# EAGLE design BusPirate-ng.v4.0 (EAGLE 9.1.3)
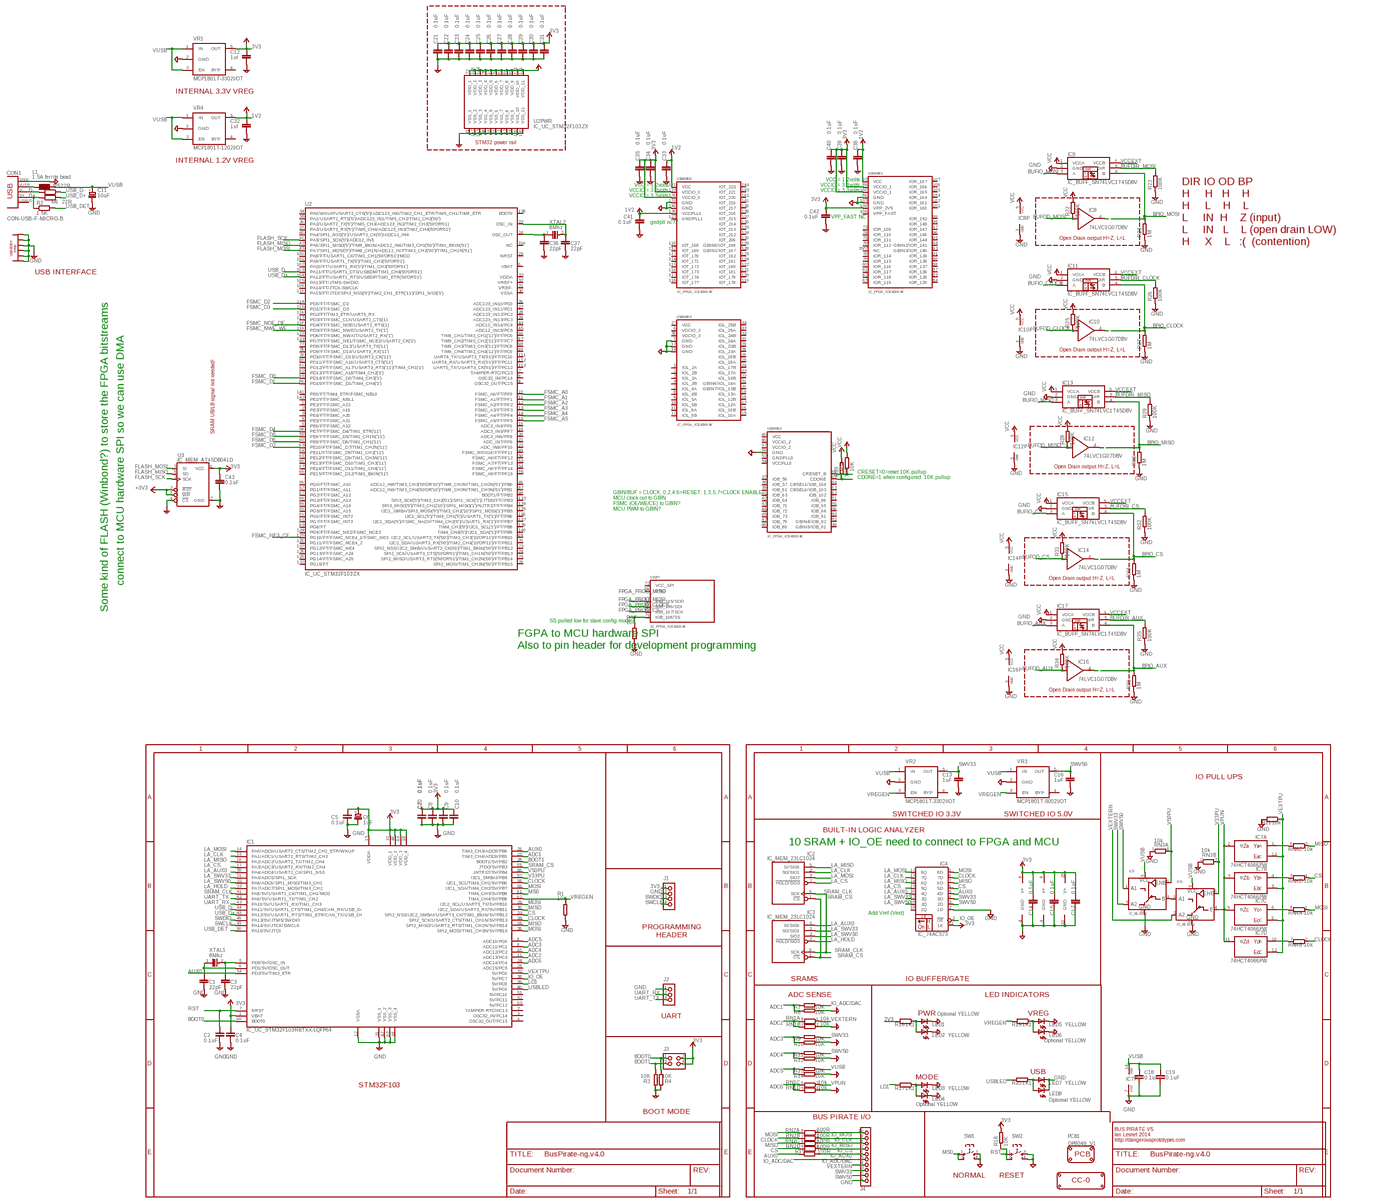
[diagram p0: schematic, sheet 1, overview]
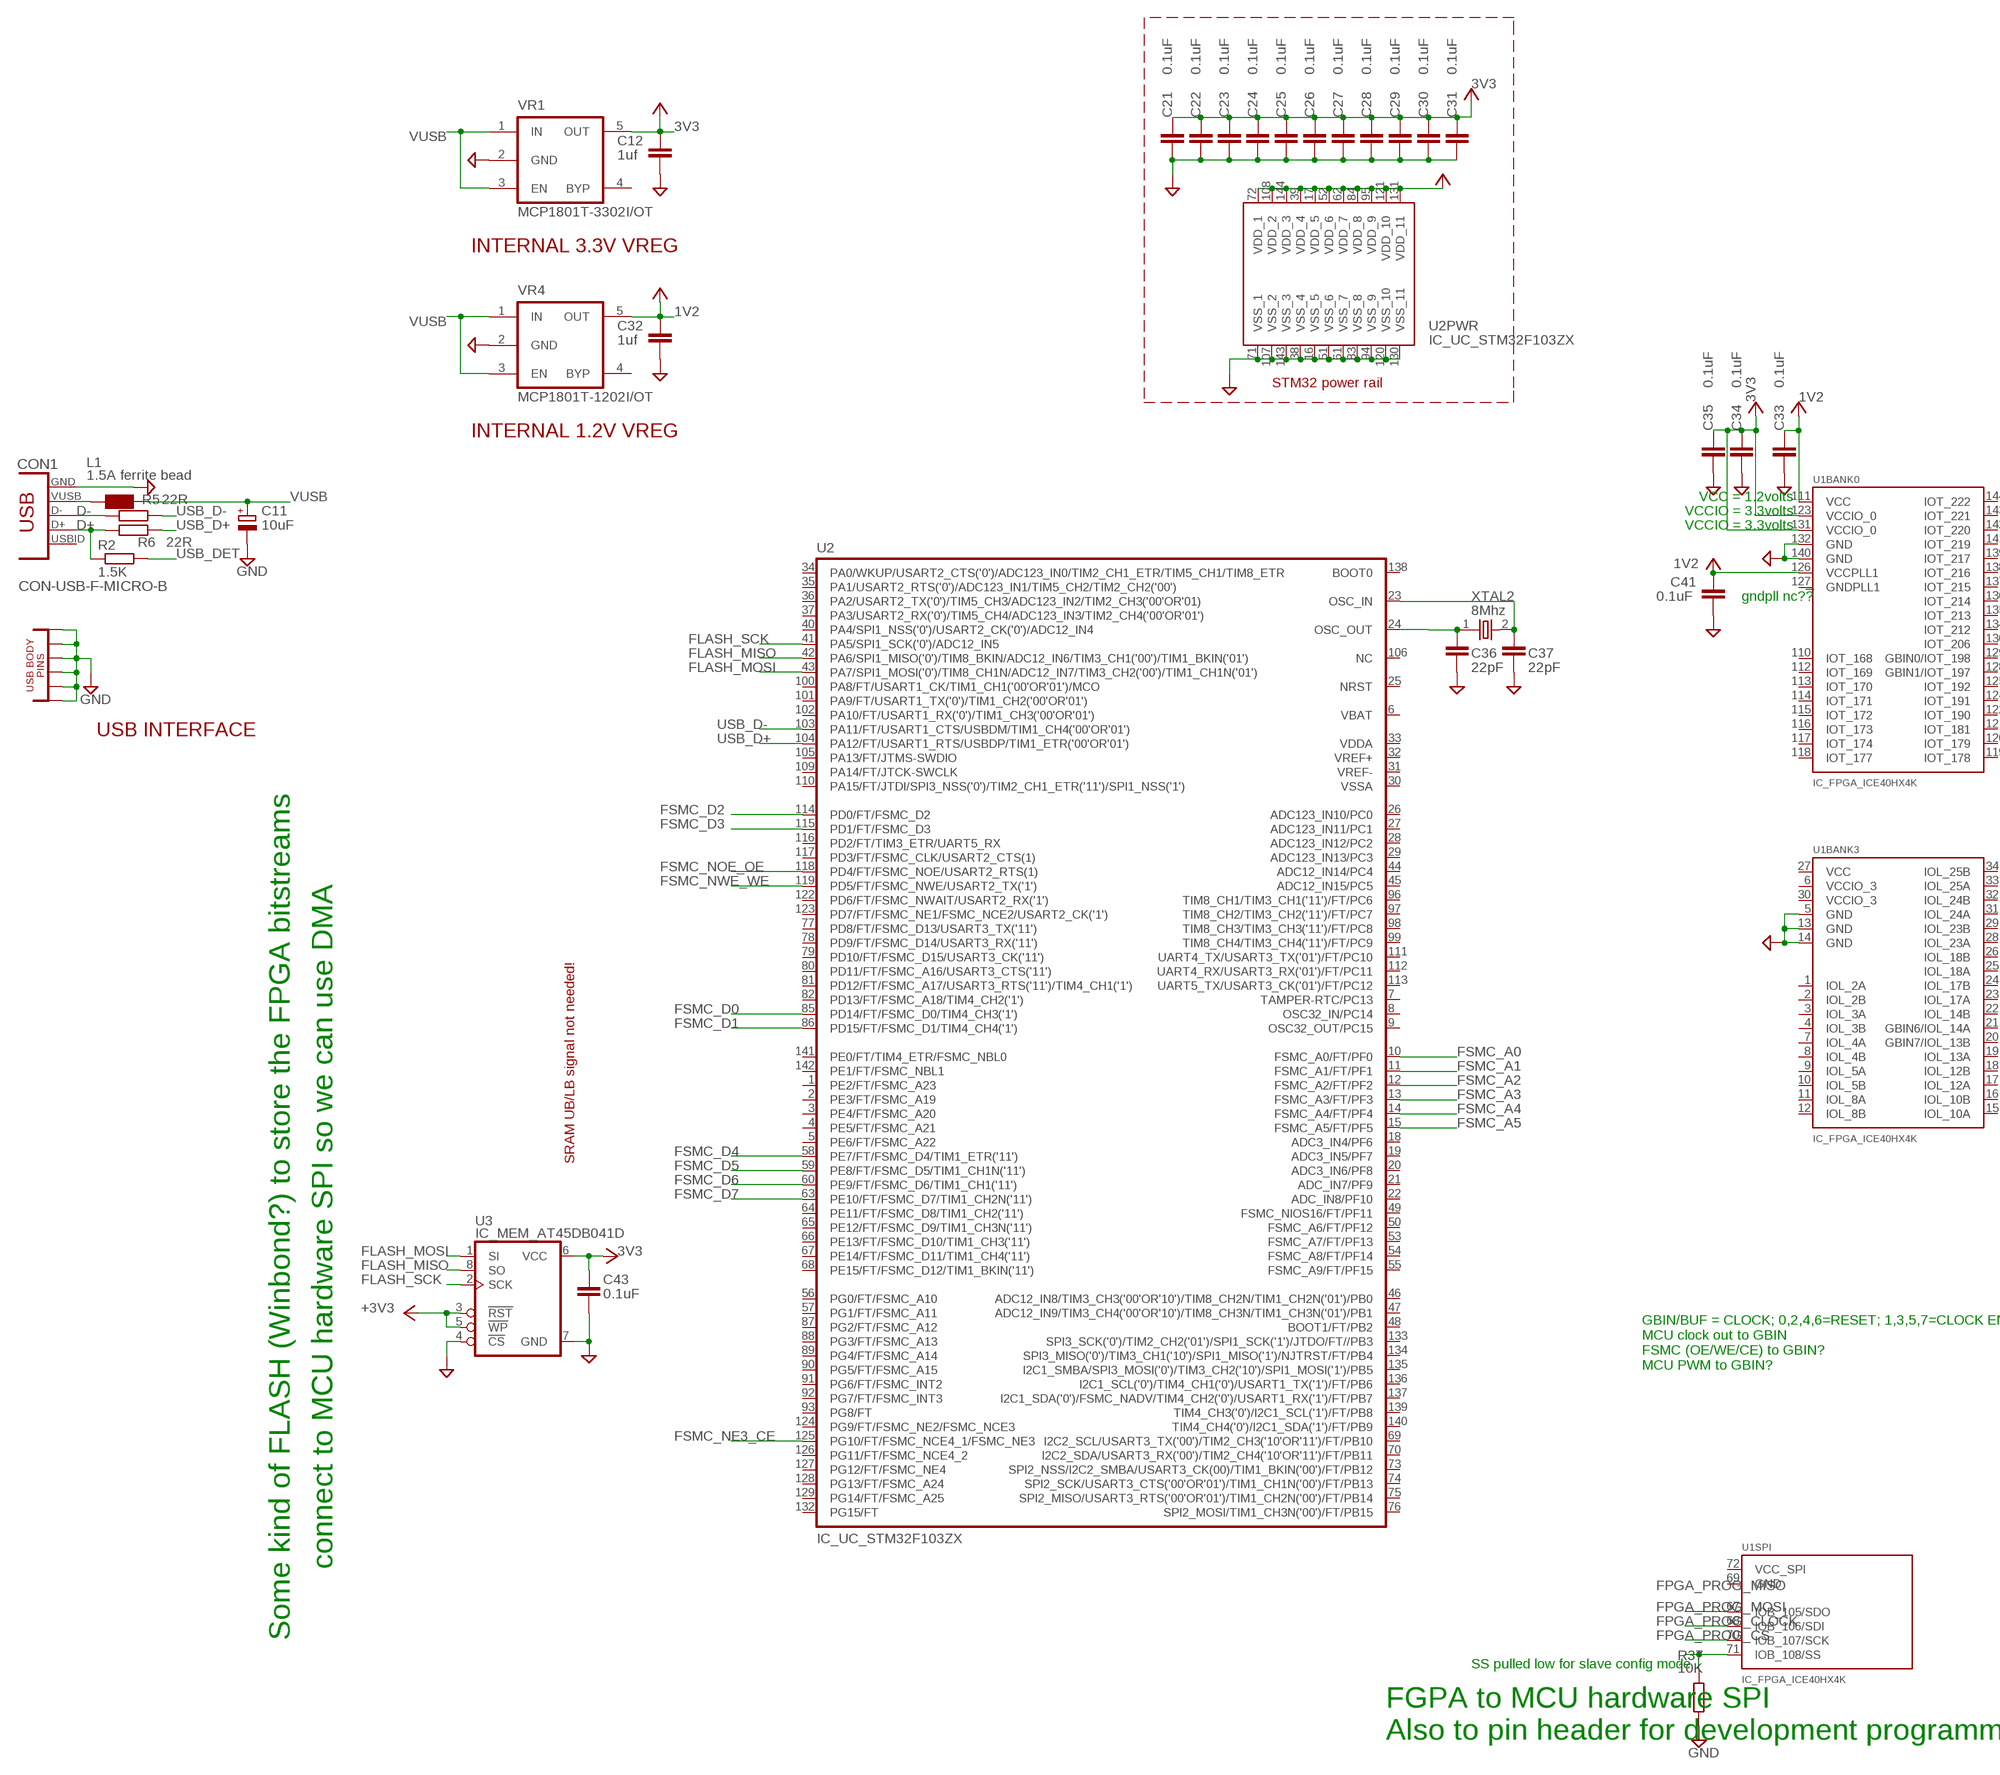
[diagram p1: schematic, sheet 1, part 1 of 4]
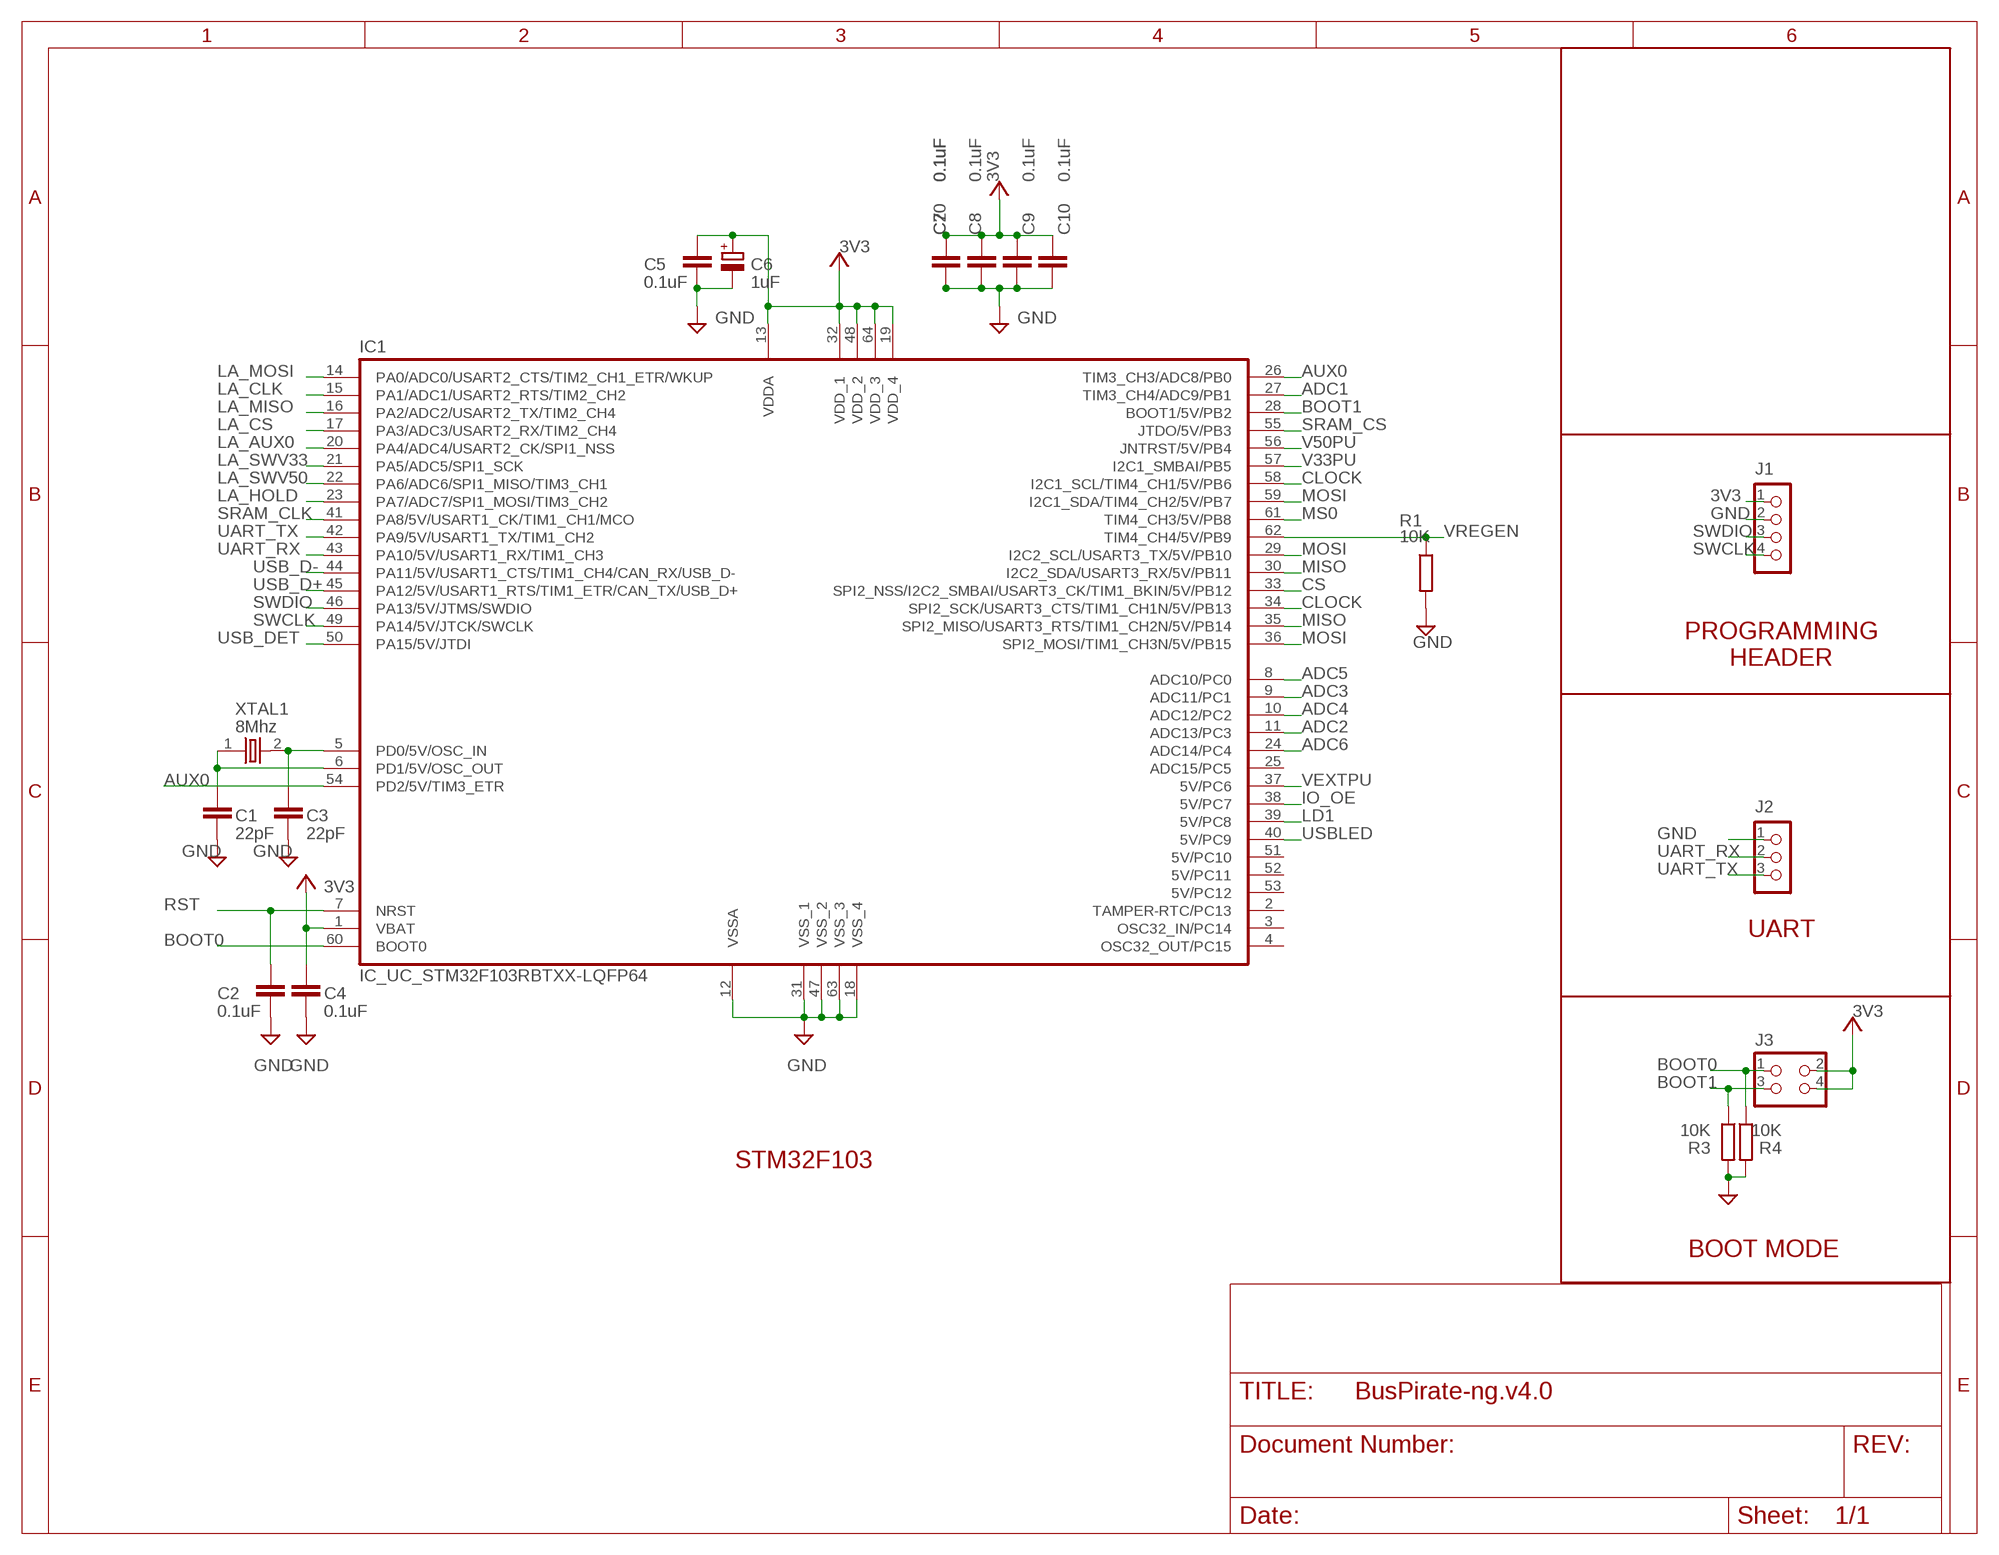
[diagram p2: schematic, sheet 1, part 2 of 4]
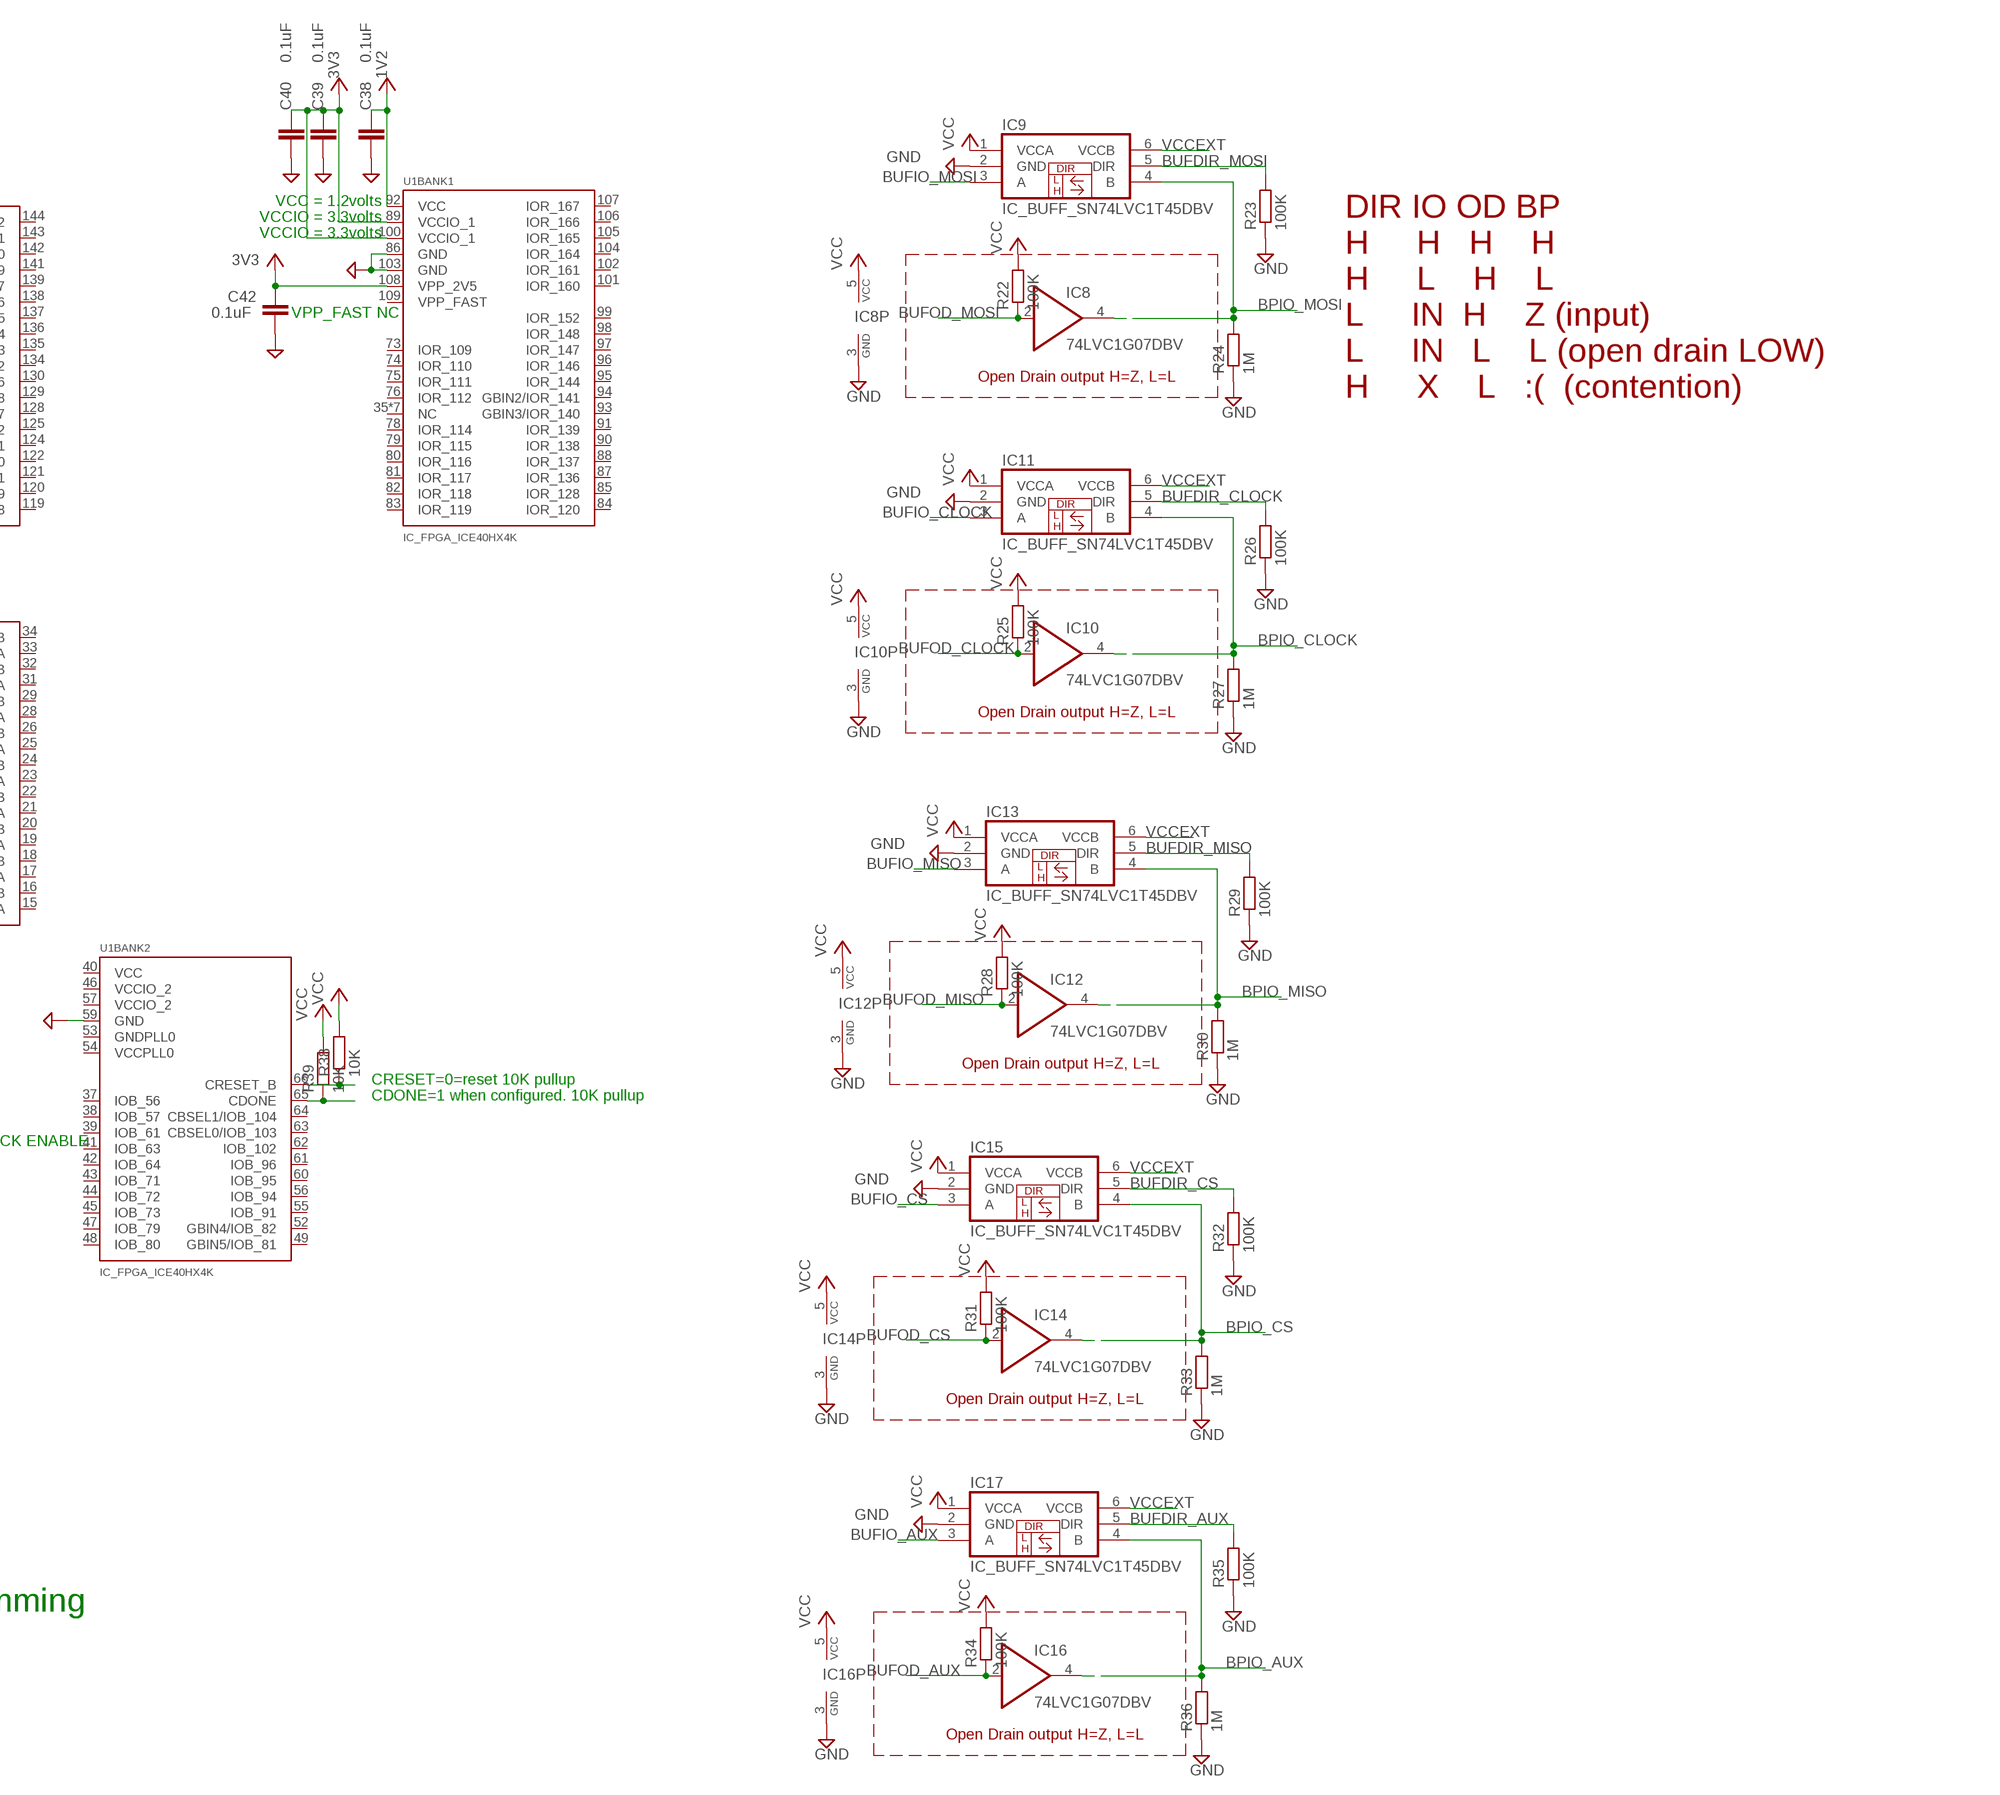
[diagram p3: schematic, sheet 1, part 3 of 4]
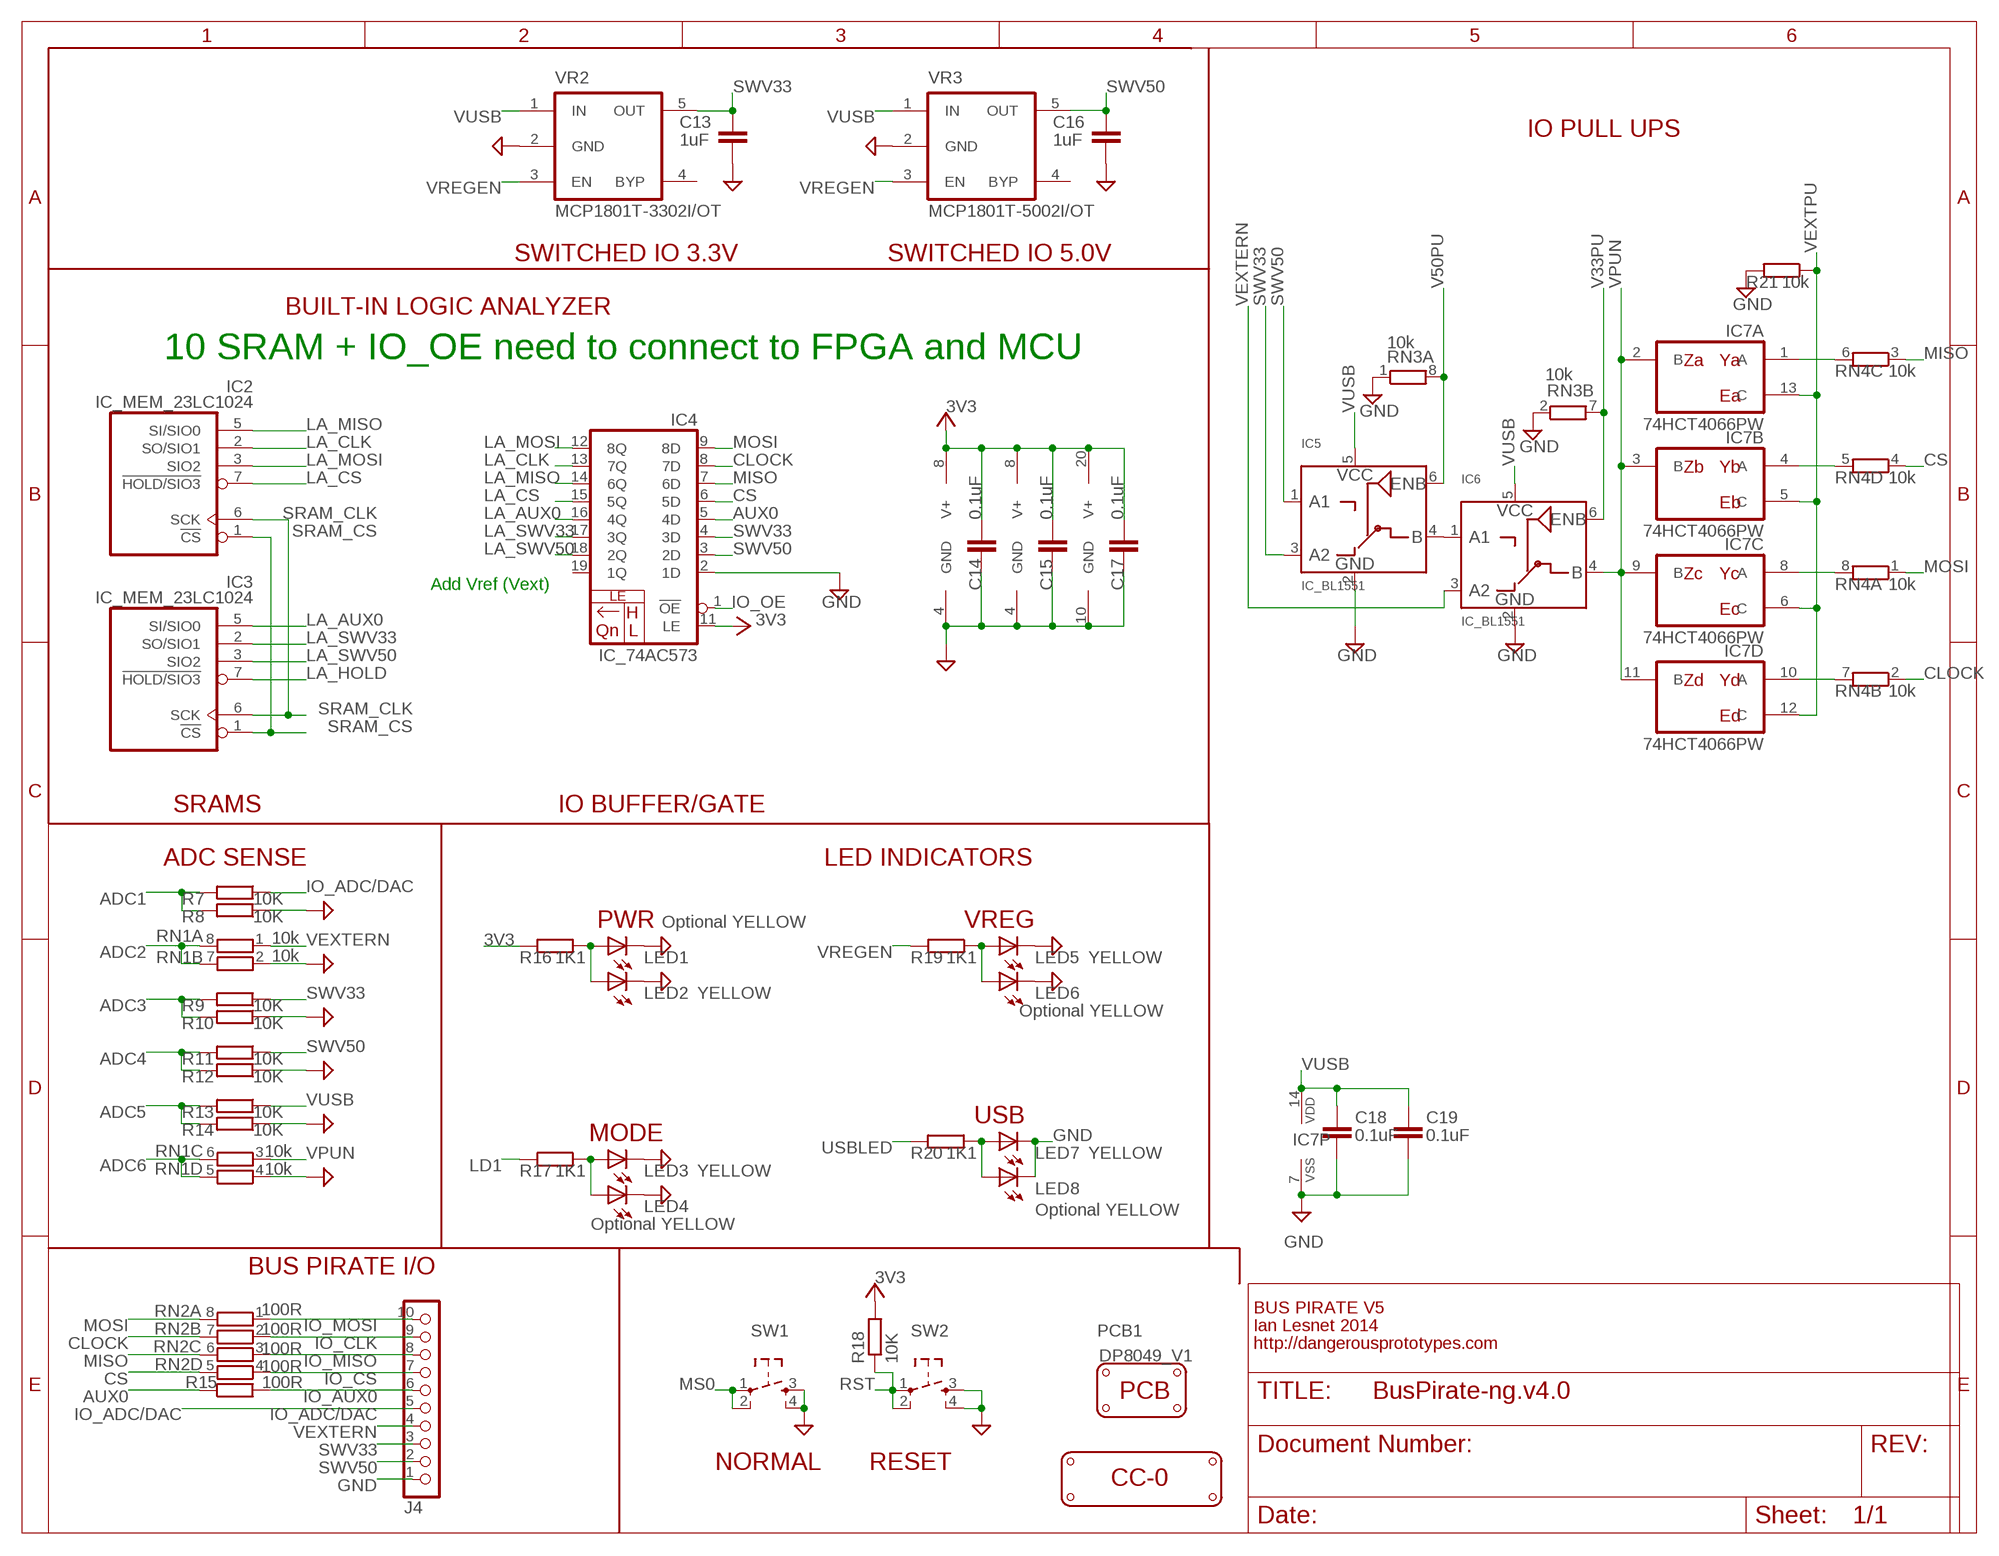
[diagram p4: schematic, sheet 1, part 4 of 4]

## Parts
C1  22pF  C-EUC0603  [C0603]
C2  0.1uF  C-EUC0603  [C0603]
C3  22pF  C-EUC0603  [C0603]
C4  0.1uF  C-EUC0603  [C0603]
C5  0.1uF  C-EUC0603  [C0603]
C6  1uF  CPOL-EUSMCA  [SMC_A]
C7  0.1uF  C-EUC0603  [C0603]
C8  0.1uF  C-EUC0603  [C0603]
C9  0.1uF  C-EUC0603  [C0603]
C10  0.1uF  C-EUC0603  [C0603]
C11  10uF  CPOL-EUSMCA  [SMC_A]
C12  1uf  C-EUC0603  [C0603]
C13  1uF  C-EUC0603  [C0603]
C14  0.1uF  C-EUC0603  [C0603]
C15  0.1uF  C-EUC0603  [C0603]
C16  1uF  C-EUC0603  [C0603]
C17  0.1uF  C-EUC0603  [C0603]
C18  0.1uF  C-EUC0603  [C0603]
C19  0.1uF  C-EUC0603  [C0603]
C20  0.1uF  C-EUC0603  [C0603]
C21  0.1uF  C-EUC0603  [C0603]
C22  0.1uF  C-EUC0603  [C0603]
C23  0.1uF  C-EUC0603  [C0603]
C24  0.1uF  C-EUC0603  [C0603]
C25  0.1uF  C-EUC0603  [C0603]
C26  0.1uF  C-EUC0603  [C0603]
C27  0.1uF  C-EUC0603  [C0603]
C28  0.1uF  C-EUC0603  [C0603]
C29  0.1uF  C-EUC0603  [C0603]
C30  0.1uF  C-EUC0603  [C0603]
C31  0.1uF  C-EUC0603  [C0603]
C32  1uf  C-EUC0603  [C0603]
C33  0.1uF  C-EUC0603  [C0603]
C34  0.1uF  C-EUC0603  [C0603]
C35  0.1uF  C-EUC0603  [C0603]
C36  22pF  C-EUC0603  [C0603]
C37  22pF  C-EUC0603  [C0603]
C38  0.1uF  C-EUC0603  [C0603]
C39  0.1uF  C-EUC0603  [C0603]
C40  0.1uF  C-EUC0603  [C0603]
C41  0.1uF  C-EUC0603  [C0603]
C42  0.1uF  C-EUC0603  [C0603]
C43  0.1uF  C-EUC0603  [C0603]
CON1  CON-USB-F-MICRO-B  [CON_USB_MICRO-B-1-MD05SMXXX-01]
IC1  IC_UC_STM32F103RBTXX-LQFP64  [LQFP64]
IC2  IC_MEM_23LC1024  [SOIC-8]
IC3  IC_MEM_23LC1024  [SOIC-8]
IC4  IC_74AC573  IC_74AC573-TSSOP-20  [TSSOP-20]
IC5  IC_BL1551  [SC-70-6]
IC6  IC_BL1551  [SC-70-6]
IC7  74HCT4066PW  4066TS  [40XX_TSSOP14]
IC8  74LVC1G07DBV  [SOT23-5]
IC9  IC_BUFF_SN74LVC1T45DBV  [DBV-R-PDSO-G6]
IC10  74LVC1G07DBV  [SOT23-5]
IC11  IC_BUFF_SN74LVC1T45DBV  [DBV-R-PDSO-G6]
IC12  74LVC1G07DBV  [SOT23-5]
IC13  IC_BUFF_SN74LVC1T45DBV  [DBV-R-PDSO-G6]
IC14  74LVC1G07DBV  [SOT23-5]
IC15  IC_BUFF_SN74LVC1T45DBV  [DBV-R-PDSO-G6]
IC16  74LVC1G07DBV  [SOT23-5]
IC17  IC_BUFF_SN74LVC1T45DBV  [DBV-R-PDSO-G6]
J1  CON_HEADER_1X04  [M1X4]
J2  CON_HEADER_1X03-PTH  [M1X3]
J3  CON_HEADER_2X02-PTH  [M2X2]
J4  CON_HEADER_1X10-RIGHT_ANGLED_PTH_SHROUDED  [M1X10_MALE_RIGHT_ANGLES_PTH_SHROUDED]
L1  1.5A ferrite bead  WE-KIL_0805  [WE-KI_0805_B]
LED1  Optional YELLOW  LED-0805  [LED-805]
LED2  YELLOW  LED-0805  [LED-805]
LED3  YELLOW  LED-0805  [LED-805]
LED4  Optional YELLOW  LED-0805  [LED-805]
LED5  YELLOW  LED-0805  [LED-805]
LED6  Optional YELLOW  LED-0805  [LED-805]
LED7  YELLOW  LED-0805  [LED-805]
LED8  Optional YELLOW  LED-0805  [LED-805]
LOGO1  LOGO_CC-0  [LOGO_CC-0]
PCB1  PCB_DP_RECTANGLE-80X49  [DP8049_V1]
R1  10K  RESISTOR-0603  [R603]
R2  1.5K  RESISTOR-0603  [R603]
R3  10K  R-EU_R0603  [R0603]
R4  10K  R-EU_R0603  [R0603]
R5  22R  RESISTOR-0603  [R603]
R6  22R  RESISTOR-0603  [R603]
R7  10K  R-EU_R0603  [R0603]
R8  10K  R-EU_R0603  [R0603]
R9  10K  R-EU_R0603  [R0603]
R10  10K  R-EU_R0603  [R0603]
R11  10K  R-EU_R0603  [R0603]
R12  10K  R-EU_R0603  [R0603]
R13  10K  R-EU_R0603  [R0603]
R14  10K  R-EU_R0603  [R0603]
R15  100R  RESISTOR-0603  [R603]
R16  1K1  RESISTOR-0603  [R603]
R17  1K1  RESISTOR-0603  [R603]
R18  10K  RESISTOR-0603  [R603]
R19  1K1  RESISTOR-0603  [R603]
R20  1K1  RESISTOR-0603  [R603]
R21  10k  RESISTOR-0603  [R603]
R22  100K  R-EU_R0603  [R0603]
R23  100K  R-EU_R0603  [R0603]
R24  1M  R-EU_R0603  [R0603]
R25  100K  R-EU_R0603  [R0603]
R26  100K  R-EU_R0603  [R0603]
R27  1M  R-EU_R0603  [R0603]
R28  100K  R-EU_R0603  [R0603]
R29  100K  R-EU_R0603  [R0603]
R30  1M  R-EU_R0603  [R0603]
R31  100K  R-EU_R0603  [R0603]
R32  100K  R-EU_R0603  [R0603]
R33  1M  R-EU_R0603  [R0603]
R34  100K  R-EU_R0603  [R0603]
R35  100K  R-EU_R0603  [R0603]
R36  1M  R-EU_R0603  [R0603]
R37  10K  RESISTOR-0603  [R603]
R38  10K  R-EU_R0603  [R0603]
R39  10K  R-EU_R0603  [R0603]
RN1  10k  RNETWORK  [RN8P-4R-CRA06S]
RN2  100R  RNETWORK  [RN8P-4R-CRA06S]
RN3  10k  RNETWORK  [RN8P-4R-CRA06S]
RN4  10k  RNETWORK  [RN8P-4R-CRA06S]
SW1  SW_TACT_4P  [SW_TACT_SMALL]
SW2  SW_TACT_4P  [SW_TACT_SMALL]
U1  IC_FPGA_ICE40HX4K  [TQFP-144]
U2  IC_UC_STM32F103ZX  [TQFP-144]
U3  IC_MEM_AT45DB041D  [SOIC-8]
VR1  MCP1801T-3302I/OT  MIC5205  [SOT-23-5@1]
VR2  MCP1801T-3302I/OT  MIC5205  [SOT-23-5@1]
VR3  MCP1801T-5002I/OT  MIC5205  [SOT-23-5@1]
VR4  MCP1801T-1202I/OT  MIC5205  [SOT-23-5@1]
XTAL1  8Mhz  OSC-XTAL-12M  [XTAL_4X6]
XTAL2  8Mhz  OSC-XTAL-12M  [XTAL_4X6]

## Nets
1V2: C32.1 C33.2 C38.2 C41.2 U1.92(BANK1:VCC) U1.111(BANK0:VCC) U1.126(BANK0:VCCPLL1) VR4.5(OUT) ; supply symbol labelled SUPPLY_+3V3
3V3: C4.2 C5.2 C6.+ C7.2 C8.2 C9.2 C10.2 C12.1 C14.1 C15.1 C17.1 C20.2 C21.2 C22.2 C23.2 C24.2 C25.2 C26.2 C27.2 C28.2 C29.2 C30.2 C31.2 C34.2 C35.2 C39.2 C40.2 C42.2 C43.2 IC1.1(VBAT) IC1.13(VDDA) IC1.19(VDD_4) IC1.32(VDD_1) IC1.48(VDD_2) IC1.64(VDD_3) IC2.8(V+) IC3.8(V+) IC4.11(LE) IC4.20(V+) J1.1 J3.2 J3.4 R16.2 R18.2 U1.89(BANK1:VCCIO_1) U1.100(BANK1:VCCIO_1) U1.108(BANK1:VPP_2V5) U1.123(BANK0:VCCIO_0) U1.131(BANK0:VCCIO_0) U2.17(VDD_5) U2.39(VDD_4) U2.52(VDD_6) U2.62(VDD_7) U2.72(VDD_1) U2.84(VDD_8) U2.95(VDD_9) U2.108(VDD_2) U2.121(VDD_10) U2.131(VDD_11) U2.144(VDD_3) U3.6(VCC) VR1.5(OUT) ; supply symbol labelled V+, SUPPLY_+3V3
+3V3: U3.3(!RST) U3.5(!WP) ; supply symbol labelled SUPPLY_+3V3
ADC1: IC1.27(TIM3_CH4/ADC9/PB1) R7.2 R8.2
ADC2: IC1.11(ADC13/PC3) RN1.7 RN1.8
ADC3: IC1.9(ADC11/PC1) R9.2 R10.2
ADC4: IC1.10(ADC12/PC2) R11.2 R12.2
ADC5: IC1.8(ADC10/PC0) R13.2 R14.2
ADC6: IC1.24(ADC14/PC4) RN1.5 RN1.6
AUX0: IC1.26(TIM3_CH3/ADC8/PB0) IC1.54(PD2/5V/TIM3_ETR) IC4.5(4D) R15.1
BOOT0: IC1.60(BOOT0) J3.1 R4.1
BOOT1: IC1.28(BOOT1/5V/PB2) J3.3 R3.1
BPIO_AUX: IC16.4(O) IC17.4(B) R36.2
BPIO_CLOCK: IC10.4(O) IC11.4(B) R27.2
BPIO_CS: IC14.4(O) IC15.4(B) R33.2
BPIO_MISO: IC12.4(O) IC13.4(B) R30.2
BPIO_MOSI: IC8.4(O) IC9.4(B) R24.2
BUFDIR_AUX: IC17.5(DIR) R35.2
BUFDIR_CLOCK: IC11.5(DIR) R26.2
BUFDIR_CS: IC15.5(DIR) R32.2
BUFDIR_MISO: IC13.5(DIR) R29.2
BUFDIR_MOSI: IC9.5(DIR) R23.2
BUFIO_AUX: IC17.3(A)
BUFIO_CLOCK: IC11.3(A)
BUFIO_CS: IC15.3(A)
BUFIO_MISO: IC13.3(A)
BUFIO_MOSI: IC9.3(A)
BUFOD_AUX: IC16.2(I) R34.1
BUFOD_CLOCK: IC10.2(I) R25.1
BUFOD_CS: IC14.2(I) R31.1
BUFOD_MISO: IC12.2(I) R28.1
BUFOD_MOSI: IC8.2(I) R22.1
CLOCK: IC1.34(SPI2_SCK/USART3_CTS/TIM1_CH1N/5V/PB13) IC1.58(I2C1_SCL/TIM4_CH1/5V/PB6) IC4.8(7D) RN2.7 RN4.2
CS: IC1.33(SPI2_NSS/I2C2_SMBAI/USART3_CK/TIM1_BKIN/5V/PB12) IC4.6(5D) RN2.5 RN4.4
D+: CON1.P3(D+) R2.1 R6.2
D-: CON1.P2(D-) R5.2
EXVUSB: CON1.P1(VUSB) L1.2
FLASH_MISO: U2.42(PA6/SPI1_MISO('0')/TIM8_BKIN/ADC12_IN6/TIM3_CH1('00')/TIM1_BKIN('01')) U3.8(SO)
FLASH_MOSI: U2.43(PA7/SPI1_MOSI('0')/TIM8_CH1N/ADC12_IN7/TIM3_CH2('00')/TIM1_CH1N('01')) U3.1(SI)
FLASH_SCK: U2.41(PA5/SPI1_SCK('0')/ADC12_IN5) U3.2(SCK)
FPGA_PROG_CLOCK: U1.70(SPI:IOB_107/SCK)
FPGA_PROG_CS: R37.1 U1.71(SPI:IOB_108/SS)
FPGA_PROG_MISO: U1.67(SPI:IOB_105/SDO)
FPGA_PROG_MOSI: U1.68(SPI:IOB_106/SDI)
FSMC_A0: U2.10(FSMC_A0/FT/PF0)
FSMC_A1: U2.11(FSMC_A1/FT/PF1)
FSMC_A2: U2.12(FSMC_A2/FT/PF2)
FSMC_A3: U2.13(FSMC_A3/FT/PF3)
FSMC_A4: U2.14(FSMC_A4/FT/PF4)
FSMC_A5: U2.15(FSMC_A5/FT/PF5)
FSMC_D0: U2.85(PD14/FT/FSMC_D0/TIM4_CH3('1'))
FSMC_D1: U2.86(PD15/FT/FSMC_D1/TIM4_CH4('1'))
FSMC_D2: U2.114(PD0/FT/FSMC_D2)
FSMC_D3: U2.115(PD1/FT/FSMC_D3)
FSMC_D4: U2.58(PE7/FT/FSMC_D4/TIM1_ETR('11'))
FSMC_D5: U2.59(PE8/FT/FSMC_D5/TIM1_CH1N('11'))
FSMC_D6: U2.60(PE9/FT/FSMC_D6/TIM1_CH1('11'))
FSMC_D7: U2.63(PE10/FT/FSMC_D7/TIM1_CH2N('11'))
FSMC_NE3_CE: U2.125(PG10/FT/FSMC_NCE4_1/FSMC_NE3)
FSMC_NOE_OE: U2.118(PD4/FT/FSMC_NOE/USART2_RTS(1))
FSMC_NWE_WE: U2.119(PD5/FT/FSMC_NWE/USART2_TX('1'))
GND: C1.1 C2.1 C3.1 C4.1 C5.1 C6.- C7.1 C8.1 C9.1 C10.1 C11.- C12.2 C13.2 C14.2 C15.2 C16.2 C17.2 C18.2 C19.2 C20.1 C21.1 C22.1 C23.1 C24.1 C25.1 C26.1 C27.1 C28.1 C29.1 C30.1 C31.1 C32.2 C33.1 C34.1 C35.1 C36.1 C37.1 C38.1 C39.1 C40.1 C41.1 C42.1 C43.1 CON1.GND1 CON1.GND2 CON1.GND3 CON1.GND4 CON1.GND5 CON1.GND6 CON1.P5(GND) IC1.12(VSSA) IC1.18(VSS_4) IC1.31(VSS_1) IC1.47(VSS_2) IC1.63(VSS_3) IC2.4(GND) IC3.4(GND) IC4.2(1D) IC4.10(GND) IC5.2(GND) IC6.2(GND) IC7.7(P:VSS) IC8.3(GND) IC9.2(GND) IC10.3(GND) IC11.2(GND) IC12.3(GND) IC13.2(GND) IC14.3(GND) IC15.2(GND) IC16.3(GND) IC17.2(GND) J1.2 J2.1 J4.1 LED1.C LED2.C LED3.C LED4.C LED5.C LED6.C LED7.C LED8.C R1.2 R3.2 R4.2 R8.1 R10.1 R12.1 R14.1 R21.2 R23.1 R24.1 R26.1 R27.1 R29.1 R30.1 R32.1 R33.1 R35.1 R36.1 R37.2 RN1.2 RN1.4 RN3.1 RN3.2 SW1.3 SW1.4 SW2.3 SW2.4 U1.5(BANK3:GND) U1.13(BANK3:GND) U1.14(BANK3:GND) U1.59(BANK2:GND) U1.86(BANK1:GND) U1.103(BANK1:GND) U1.132(BANK0:GND) U1.140(BANK0:GND) U2.16(VSS_5) U2.38(VSS_4) U2.51(VSS_6) U2.61(VSS_7) U2.71(VSS_1) U2.83(VSS_8) U2.94(VSS_9) U2.107(VSS_2) U2.120(VSS_10) U2.130(VSS_11) U2.143(VSS_3) U3.4(!CS) U3.7(GND) VR1.2(GND) VR2.2(GND) VR3.2(GND) VR4.2(GND)
IO_ADC/DAC: J4.5 R7.1
IO_AUX0: J4.6 R15.2
IO_CLK: J4.9 RN2.2
IO_CS: J4.7 RN2.4
IO_MISO: J4.8 RN2.3
IO_MOSI: J4.10 RN2.1
IO_OE: IC1.38(5V/PC7) IC4.1(!OE)
LA_AUX0: IC1.20(PA4/ADC4/USART2_CK/SPI1_NSS) IC3.5(SI/SIO0) IC4.16(4Q)
LA_CLK: IC1.15(PA1/ADC1/USART2_RTS/TIM2_CH2) IC2.2(SO/SIO1) IC4.13(7Q)
LA_CS: IC1.17(PA3/ADC3/USART2_RX/TIM2_CH4) IC2.7(!HOLD/SIO3) IC4.15(5Q)
LA_HOLD: IC1.23(PA7/ADC7/SPI1_MOSI/TIM3_CH2) IC3.7(!HOLD/SIO3)
LA_MISO: IC1.16(PA2/ADC2/USART2_TX/TIM2_CH4) IC2.5(SI/SIO0) IC4.14(6Q)
LA_MOSI: IC1.14(PA0/ADC0/USART2_CTS/TIM2_CH1_ETR/WKUP) IC2.3(SIO2) IC4.12(8Q)
LA_SWV33: IC1.21(PA5/ADC5/SPI1_SCK) IC3.2(SO/SIO1) IC4.17(3Q)
LA_SWV50: IC1.22(PA6/ADC6/SPI1_MISO/TIM3_CH1) IC3.3(SIO2) IC4.18(2Q)
LD1: IC1.39(5V/PC8) R17.2
MISO: IC1.30(I2C2_SDA/USART3_RX/5V/PB11) IC1.35(SPI2_MISO/USART3_RTS/TIM1_CH2N/5V/PB14) IC4.7(6D) RN2.6 RN4.3
MOSI: IC1.29(I2C2_SCL/USART3_TX/5V/PB10) IC1.36(SPI2_MOSI/TIM1_CH3N/5V/PB15) IC1.59(I2C1_SDA/TIM4_CH2/5V/PB7) IC4.9(8D) RN2.8 RN4.1
MS0: IC1.61(TIM4_CH3/5V/PB8) SW1.1 SW1.2
N$1: IC5.4(B) IC6.1(A1)
N$2: IC7.1(A:A) RN4.6
N$3: IC7.4(B:A) RN4.5
N$4: IC7.8(C:A) RN4.8
N$5: IC7.10(D:A) RN4.7
N$6: LED3.A LED4.A R17.1
N$7: LED1.A LED2.A R16.1
N$8: C37.2 U2.23(OSC_IN) XTAL2.2
N$9: C36.2 U2.24(OSC_OUT) XTAL2.1
N$12: R38.1 U1.66(BANK2:CRESET_B)
N$13: LED7.A LED8.A R20.1
N$14: R39.1 U1.65(BANK2:CDONE)
N$16: C3.2 IC1.5(PD0/5V/OSC_IN) XTAL1.2
N$18: LED5.A LED6.A R19.1
N$20: C1.2 IC1.6(PD1/5V/OSC_OUT) XTAL1.1
RST: C2.2 IC1.7(NRST) R18.1 SW2.1 SW2.2
SRAM_CLK: IC1.41(PA8/5V/USART1_CK/TIM1_CH1/MCO) IC2.6(SCK) IC3.6(SCK)
SRAM_CS: IC1.55(JTDO/5V/PB3) IC2.1(!CS) IC3.1(!CS)
SWCLK: IC1.49(PA14/5V/JTCK/SWCLK) J1.4
SWDIO: IC1.46(PA13/5V/JTMS/SWDIO) J1.3
SWV33: C13.1 IC4.4(3D) IC5.3(A2) J4.3 R9.1 VR2.5(OUT)
SWV50: C16.1 IC4.3(2D) IC5.1(A1) J4.2 R11.1 VR3.5(OUT)
UART_RX: IC1.43(PA10/5V/USART1_RX/TIM1_CH3) J2.2
UART_TX: IC1.42(PA9/5V/USART1_TX/TIM1_CH2) J2.3
USB_D+: IC1.45(PA12/5V/USART1_RTS/TIM1_ETR/CAN_TX/USB_D+) R6.1 U2.104(PA12/FT/USART1_RTS/USBDP/TIM1_ETR('00'OR'01'))
USB_D-: IC1.44(PA11/5V/USART1_CTS/TIM1_CH4/CAN_RX/USB_D-) R5.1 U2.103(PA11/FT/USART1_CTS/USBDM/TIM1_CH4('00'OR'01'))
USB_DET: IC1.50(PA15/5V/JTDI) R2.2
USBLED: IC1.40(5V/PC9) R20.2
V33PU: IC1.57(I2C1_SMBAI/PB5) IC6.6(ENB) RN3.7
V50PU: IC1.56(JNTRST/5V/PB4) IC5.6(ENB) RN3.8
VCC: IC8.5(VCC) IC9.1(VCCA) IC10.5(VCC) IC11.1(VCCA) IC12.5(VCC) IC13.1(VCCA) IC14.5(VCC) IC15.1(VCCA) IC16.5(VCC) IC17.1(VCCA) R22.2 R25.2 R28.2 R31.2 R34.2 R38.2 R39.2
VCCEXT: IC9.6(VCCB) IC11.6(VCCB) IC13.6(VCCB) IC15.6(VCCB) IC17.6(VCCB)
VEXTERN: IC6.3(A2) J4.4 RN1.1
VEXTPU: IC1.37(5V/PC6) IC7.5(B:C) IC7.6(C:C) IC7.12(D:C) IC7.13(A:C) R21.1
VPUN: IC6.4(B) IC7.2(A:B) IC7.3(B:B) IC7.9(C:B) IC7.11(D:B) RN1.3
VREGEN: IC1.62(TIM4_CH4/5V/PB9) R1.1 R19.2 VR2.3(EN) VR3.3(EN)
VUSB: C11.+ C18.1 C19.1 IC5.5(VCC) IC6.5(VCC) IC7.14(P:VDD) L1.1 R13.1 VR1.1(IN) VR1.3(EN) VR2.1(IN) VR3.1(IN) VR4.1(IN) VR4.3(EN)
Unconnected: CON1.P4(USBID) IC1.2(TAMPER-RTC/PC13) IC1.3(OSC32_IN/PC14) IC1.4(OSC32_OUT/PC15) IC1.25(ADC15/PC5) IC1.51(5V/PC10) IC1.52(5V/PC11) IC1.53(5V/PC12) IC4.19(1Q) RN3.3 RN3.4 RN3.5 RN3.6 U1.1(BANK3:IOL_2A) U1.2(BANK3:IOL_2B) U1.3(BANK3:IOL_3A) U1.4(BANK3:IOL_3B) U1.7(BANK3:IOL_4A) U1.8(BANK3:IOL_4B) U1.9(BANK3:IOL_5A) U1.10(BANK3:IOL_5B) U1.11(BANK3:IOL_8A) U1.12(BANK3:IOL_8B) U1.15(BANK3:IOL_10A) U1.16(BANK3:IOL_10B) U1.17(BANK3:IOL_12A) U1.18(BANK3:IOL_12B) U1.19(BANK3:IOL_13A) U1.20(BANK3:GBIN7/IOL_13B) U1.21(BANK3:GBIN6/IOL_14A) U1.22(BANK3:IOL_14B) U1.23(BANK3:IOL_17A) U1.24(BANK3:IOL_17B) U1.25(BANK3:IOL_18A) U1.26(BANK3:IOL_18B) U1.28(BANK3:IOL_23A) U1.29(BANK3:IOL_23B) U1.31(BANK3:IOL_24A) U1.32(BANK3:IOL_24B) U1.33(BANK3:IOL_25A) U1.34(BANK3:IOL_25B) U1.35(BANK1:NC) U1.36(BANK1:NC) U1.37(BANK2:IOB_56) U1.38(BANK2:IOB_57) U1.39(BANK2:IOB_61) U1.41(BANK2:IOB_63) U1.42(BANK2:IOB_64) U1.43(BANK2:IOB_71) U1.44(BANK2:IOB_72) U1.45(BANK2:IOB_73) U1.47(BANK2:IOB_79) U1.48(BANK2:IOB_80) U1.49(BANK2:GBIN5/IOB_81) U1.50(BANK1:NC) U1.51(BANK1:NC) U1.52(BANK2:GBIN4/IOB_82) U1.55(BANK2:IOB_91) U1.56(BANK2:IOB_94) U1.58(BANK1:NC) U1.60(BANK2:IOB_95) U1.61(BANK2:IOB_96) U1.62(BANK2:IOB_102) U1.63(BANK2:CBSEL0/IOB_103) U1.64(BANK2:CBSEL1/IOB_104) U1.73(BANK1:IOR_109) U1.74(BANK1:IOR_110) U1.75(BANK1:IOR_111) U1.76(BANK1:IOR_112) U1.77(BANK1:NC) U1.78(BANK1:IOR_114) U1.79(BANK1:IOR_115) U1.80(BANK1:IOR_116) U1.81(BANK1:IOR_117) U1.82(BANK1:IOR_118) U1.83(BANK1:IOR_119) U1.84(BANK1:IOR_120) U1.85(BANK1:IOR_128) U1.87(BANK1:IOR_136) U1.88(BANK1:IOR_137) U1.90(BANK1:IOR_138) U1.91(BANK1:IOR_139) U1.93(BANK1:GBIN3/IOR_140) U1.94(BANK1:GBIN2/IOR_141) U1.95(BANK1:IOR_144) U1.96(BANK1:IOR_146) U1.97(BANK1:IOR_147) U1.98(BANK1:IOR_148) U1.99(BANK1:IOR_152) U1.101(BANK1:IOR_160) U1.102(BANK1:IOR_161) U1.104(BANK1:IOR_164) U1.105(BANK1:IOR_165) U1.106(BANK1:IOR_166) U1.107(BANK1:IOR_167) U1.110(BANK0:IOT_168) U1.112(BANK0:IOT_169) U1.113(BANK0:IOT_170) U1.114(BANK0:IOT_171) U1.115(BANK0:IOT_172) U1.116(BANK0:IOT_173) U1.117(BANK0:IOT_174) U1.118(BANK0:IOT_177) U1.119(BANK0:IOT_178) U1.120(BANK0:IOT_179) U1.121(BANK0:IOT_181) U1.122(BANK0:IOT_190) U1.124(BANK0:IOT_191) U1.125(BANK0:IOT_192) U1.128(BANK0:GBIN1/IOT_197) U1.129(BANK0:GBIN0/IOT_198) U1.130(BANK0:IOT_206) U1.133(BANK1:NC) U1.134(BANK0:IOT_212) U1.135(BANK0:IOT_213) U1.136(BANK0:IOT_214) U1.137(BANK0:IOT_215) U1.138(BANK0:IOT_216) U1.139(BANK0:IOT_217) U1.141(BANK0:IOT_219) U1.142(BANK0:IOT_220) U1.143(BANK0:IOT_221) U1.144(BANK0:IOT_222) U2.1(PE2/FT/FSMC_A23) U2.2(PE3/FT/FSMC_A19) U2.3(PE4/FT/FSMC_A20) U2.4(PE5/FT/FSMC_A21) U2.5(PE6/FT/FSMC_A22) U2.6(VBAT) U2.7(TAMPER-RTC/PC13) U2.8(OSC32_IN/PC14) U2.9(OSC32_OUT/PC15) U2.18(ADC3_IN4/PF6) U2.19(ADC3_IN5/PF7) U2.20(ADC3_IN6/PF8) U2.21(ADC_IN7/PF9) U2.22(ADC_IN8/PF10) U2.25(NRST) U2.26(ADC123_IN10/PC0) U2.27(ADC123_IN11/PC1) U2.28(ADC123_IN12/PC2) U2.29(ADC123_IN13/PC3) U2.30(VSSA) U2.31(VREF-) U2.32(VREF+) U2.33(VDDA) U2.34(PA0/WKUP/USART2_CTS('0')/ADC123_IN0/TIM2_CH1_ETR/TIM5_CH1/TIM8_ETR) U2.35(PA1/USART2_RTS('0')/ADC123_IN1/TIM5_CH2/TIM2_CH2('00')) U2.36(PA2/USART2_TX('0')/TIM5_CH3/ADC123_IN2/TIM2_CH3('00'OR'01)) U2.37(PA3/USART2_RX('0')/TIM5_CH4/ADC123_IN3/TIM2_CH4('00'OR'01')) U2.40(PA4/SPI1_NSS('0')/USART2_CK('0')/ADC12_IN4) U2.44(ADC12_IN14/PC4) U2.45(ADC12_IN15/PC5) U2.46(ADC12_IN8/TIM3_CH3('00'OR'10')/TIM8_CH2N/TIM1_CH2N('01')/PB0) U2.47(ADC12_IN9/TIM3_CH4('00'OR'10')/TIM8_CH3N/TIM1_CH3N('01')/PB1) U2.48(BOOT1/FT/PB2) U2.49(FSMC_NIOS16/FT/PF11) U2.50(FSMC_A6/FT/PF12) U2.53(FSMC_A7/FT/PF13) U2.54(FSMC_A8/FT/PF14) U2.55(FSMC_A9/FT/PF15) U2.56(PG0/FT/FSMC_A10) U2.57(PG1/FT/FSMC_A11) U2.64(PE11/FT/FSMC_D8/TIM1_CH2('11')) U2.65(PE12/FT/FSMC_D9/TIM1_CH3N('11')) U2.66(PE13/FT/FSMC_D10/TIM1_CH3('11')) U2.67(PE14/FT/FSMC_D11/TIM1_CH4('11')) U2.68(PE15/FT/FSMC_D12/TIM1_BKIN('11')) U2.69(I2C2_SCL/USART3_TX('00')/TIM2_CH3('10'OR'11')/FT/PB10) U2.70(I2C2_SDA/USART3_RX('00')/TIM2_CH4('10'OR'11')/FT/PB11) U2.73(SPI2_NSS/I2C2_SMBA/USART3_CK(00)/TIM1_BKIN('00')/FT/PB12) U2.74(SPI2_SCK/USART3_CTS('00'OR'01')/TIM1_CH1N('00')/FT/PB13) U2.75(SPI2_MISO/USART3_RTS('00'OR'01')/TIM1_CH2N('00')/FT/PB14) U2.76(SPI2_MOSI/TIM1_CH3N('00')/FT/PB15) U2.77(PD8/FT/FSMC_D13/USART3_TX('11')) U2.78(PD9/FT/FSMC_D14/USART3_RX('11')) U2.79(PD10/FT/FSMC_D15/USART3_CK('11')) U2.80(PD11/FT/FSMC_A16/USART3_CTS('11')) U2.81(PD12/FT/FSMC_A17/USART3_RTS('11')/TIM4_CH1('1')) U2.82(PD13/FT/FSMC_A18/TIM4_CH2('1')) U2.87(PG2/FT/FSMC_A12) U2.88(PG3/FT/FSMC_A13) U2.89(PG4/FT/FSMC_A14) U2.90(PG5/FT/FSMC_A15) U2.91(PG6/FT/FSMC_INT2) U2.92(PG7/FT/FSMC_INT3) U2.93(PG8/FT) U2.96(TIM8_CH1/TIM3_CH1('11')/FT/PC6) U2.97(TIM8_CH2/TIM3_CH2('11')/FT/PC7) U2.98(TIM8_CH3/TIM3_CH3('11')/FT/PC8) U2.99(TIM8_CH4/TIM3_CH4('11')/FT/PC9) U2.100(PA8/FT/USART1_CK/TIM1_CH1('00'OR'01')/MCO) U2.101(PA9/FT/USART1_TX('0')/TIM1_CH2('00'OR'01')) U2.102(PA10/FT/USART1_RX('0')/TIM1_CH3('00'OR'01')) U2.105(PA13/FT/JTMS-SWDIO) U2.106(NC) U2.109(PA14/FT/JTCK-SWCLK) U2.110(PA15/FT/JTDI/SPI3_NSS('0')/TIM2_CH1_ETR('11')/SPI1_NSS('1')) U2.111(UART4_TX/USART3_TX('01')/FT/PC10) U2.112(UART4_RX/USART3_RX('01')/FT/PC11) U2.113(UART5_TX/USART3_CK('01')/FT/PC12) U2.116(PD2/FT/TIM3_ETR/UART5_RX) U2.117(PD3/FT/FSMC_CLK/USART2_CTS(1)) U2.122(PD6/FT/FSMC_NWAIT/USART2_RX('1')) U2.123(PD7/FT/FSMC_NE1/FSMC_NCE2/USART2_CK('1')) U2.124(PG9/FT/FSMC_NE2/FSMC_NCE3) U2.126(PG11/FT/FSMC_NCE4_2) U2.127(PG12/FT/FSMC_NE4) U2.128(PG13/FT/FSMC_A24) U2.129(PG14/FT/FSMC_A25) U2.132(PG15/FT) U2.133(SPI3_SCK('0')/TIM2_CH2('01')/SPI1_SCK('1')/JTDO/FT//PB3) U2.134(SPI3_MISO('0')/TIM3_CH1('10')/SPI1_MISO('1')/NJTRST/FT/PB4) U2.135(I2C1_SMBA/SPI3_MOSI('0')/TIM3_CH2('10')/SPI1_MOSI('1')/PB5) U2.136(I2C1_SCL('0')/TIM4_CH1('0')/USART1_TX('1')/FT/PB6) U2.137(I2C1_SDA('0')/FSMC_NADV/TIM4_CH2('0')/USART1_RX('1')/FT/PB7) U2.138(BOOT0) U2.139(TIM4_CH3('0')/I2C1_SCL('1')/FT/PB8) U2.140(TIM4_CH4('0')/I2C1_SDA('1')/FT/PB9) U2.141(PE0/FT/TIM4_ETR/FSMC_NBL0) U2.142(PE1/FT/FSMC_NBL1) VR1.4(BYP) VR2.4(BYP) VR3.4(BYP) VR4.4(BYP)

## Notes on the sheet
- INTERNAL 3.3V VREG
- STM32 power rail
- INTERNAL 1.2V VREG
- VCC = 1.2volts
- VCC = 1.2volts | VCCIO = 3.3volts
- VCCIO = 3.3volts | VCCIO = 3.3volts
- VCCIO = 3.3volts
- VPP_FAST NC
- gndpll nc?!?
- Open Drain output H=Z, L=L
- DIR IO OD BP
  H     H   H    H
  H     L    H    L
  L     IN  H    Z (input)
  L     IN   L    L (open drain LOW)
  H     X    L   :(  (contention)
- USB INTERFACE
- Open Drain output H=Z, L=L
- SRAM UB/LB signal not needed!
- Open Drain output H=Z, L=L
- CRESET=0=reset 10K pullup
- CDONE=1 when configured. 10K pullup
- GBIN/BUF = CLOCK; 0,2,4,6=RESET; 1,3,5,7=CLOCK ENABLE
  MCU clock out to GBIN
  FSMC (OE/WE/CE) to GBIN?
  MCU PWM to GBIN?
- Open Drain output H=Z, L=L
- connect to MCU hardware SPI so we can use DMA
- Some kind of FLASH (Winbond?) to store the FPGA bitstreams
- SS pulled low for slave config mode
- FGPA to MCU hardware SPI
  Also to pin header for development programming
- Open Drain output H=Z, L=L
- IO PULL UPS
- SWITCHED IO 3.3V | SWITCHED IO 5.0V
- BUILT-IN LOGIC ANALYZER
- 10 SRAM + IO_OE need to connect to FPGA and MCU
- Za | Ya
- Ea
- Zb | Yb
- Eb
- Zc | Yc
- Add Vref (Vext)
- Ec
- PROGRAMMING
  HEADER
- Zd | Yd
- Ed
- SRAMS | IO BUFFER/GATE
- ADC SENSE | LED INDICATORS
- PWR | VREG
- UART
- USB
- MODE
- STM32F103
- BOOT MODE
- BUS PIRATE I/O
- BUS PIRATE V5
- Ian Lesnet 2014
- http://dangerousprototypes.com
- NORMAL | RESET

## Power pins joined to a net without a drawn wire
3V3: U1.27(BANK3:VCC) U1.40(BANK2:VCC)
GND: U1.69(SPI:GND)
GNDPLL0: U1.53(BANK2:GNDPLL0)
GNDPLL1: U1.127(BANK0:GNDPLL1)
VCC_SPI: U1.72(SPI:VCC_SPI)
VCCIO_2: U1.46(BANK2:VCCIO_2) U1.57(BANK2:VCCIO_2)
VCCIO_3: U1.6(BANK3:VCCIO_3) U1.30(BANK3:VCCIO_3)
VCCPLL0: U1.54(BANK2:VCCPLL0)
VPP_FAST: U1.109(BANK1:VPP_FAST)

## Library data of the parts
C1-C5 C7-C10 C12-C43 = rcl:C-EU: CAPACITOR, European symbol
C6 C11 = rcl:CPOL-EU: POLARIZED CAPACITOR, European symbol
CON1 = dp_devices.v6:CON-USB-F-MICRO-B: Micro USB 5P/F B Type SMT 1-MD05SMXXX-01
IC1 = dp_devices:IC_UC_STM32F103RBTXX: 32-bit ARM-based MCU with 64 or 128KB Flash
IC2 IC3 = dp_devices:IC_MEM_23LC1024: 1Mbit SPI SRAM with Serial dual interface and Serial quad interface
IC4 = dp_devices:IC_74AC573: 8 Transparent Latch with 3-state output Mfr no: SN74AC573NSR Digikey
IC5 IC6 = dp_devices.v6:IC_BL1551: BL1551 Low Voltage SPDT Analog Switch
IC7 = 40xx:4066: Quad bilateral ANALOG SWITCH
IC8 IC10 IC12 IC14 IC16 = 74xx-little-de:74*1G07: Single Buffer/Driver With Open-Drain Output
IC9 IC11 IC13 IC15 IC17 = dp_devices.v6:IC_BUFF_SN74LVC1T45DBV
J1 = dp_devices.v6:CON_HEADER_1X04
J2 = dp_devices.v6:CON_HEADER_1X03
J3 = dp_devices:CON_HEADER_2X02
J4 = dp_devices.v6:CON_HEADER_1X10
L1 = wuerth-elektronik:WE-KIL: SMD Wire Wound Ceramic Inductor WE-KIL
LED1-LED8 = dp_devices.v6:LED: Light Emitting Diode
LOGO1 = dp_devices:LOGO_CC-0
PCB1 = dp_devices:PCB_DP_RECTANGLE: Dangerous Prototypes Standard Rectangular PCB sizes; PCB_SIZE: DP8049_V1
R1 R16 R17 R19-R21 R37 = dp_devices:RESISTOR
R2 R5 R6 R15 R18 = dp_devices.v6:RESISTOR
R3 R4 R22-R36 R38 R39 = rcl:R-EU_: RESISTOR, European symbol
R7-R14 = resistor:R-EU_: RESISTOR, European symbol
RN1-RN4 = dp_devices:RNETWORK: 4 Resistor Array 0603
SW1 SW2 = dp_devices.v6:SW_TACT_4P
U1 = dp_devices.v6:IC_FPGA_ICE40HX4K: iCE40HX4K iCE40™ HX ultra-low power, non-volatile FPGA
U2 = dp_devices.v6:IC_UC_STM32F103ZX: STM32F103ZX High-density performance line ARM based 32-bit MCU
U3 = dp_devices.v6:IC_MEM_AT45DB041D: AT45DB041D 4-Mbit 2.5V to 3.6V Flash
VR1-VR4 = dp_devices:MIC5205: 150ma Low-Noise LDO Regulator
XTAL1 XTAL2 = dp_devices:OSC-XTAL

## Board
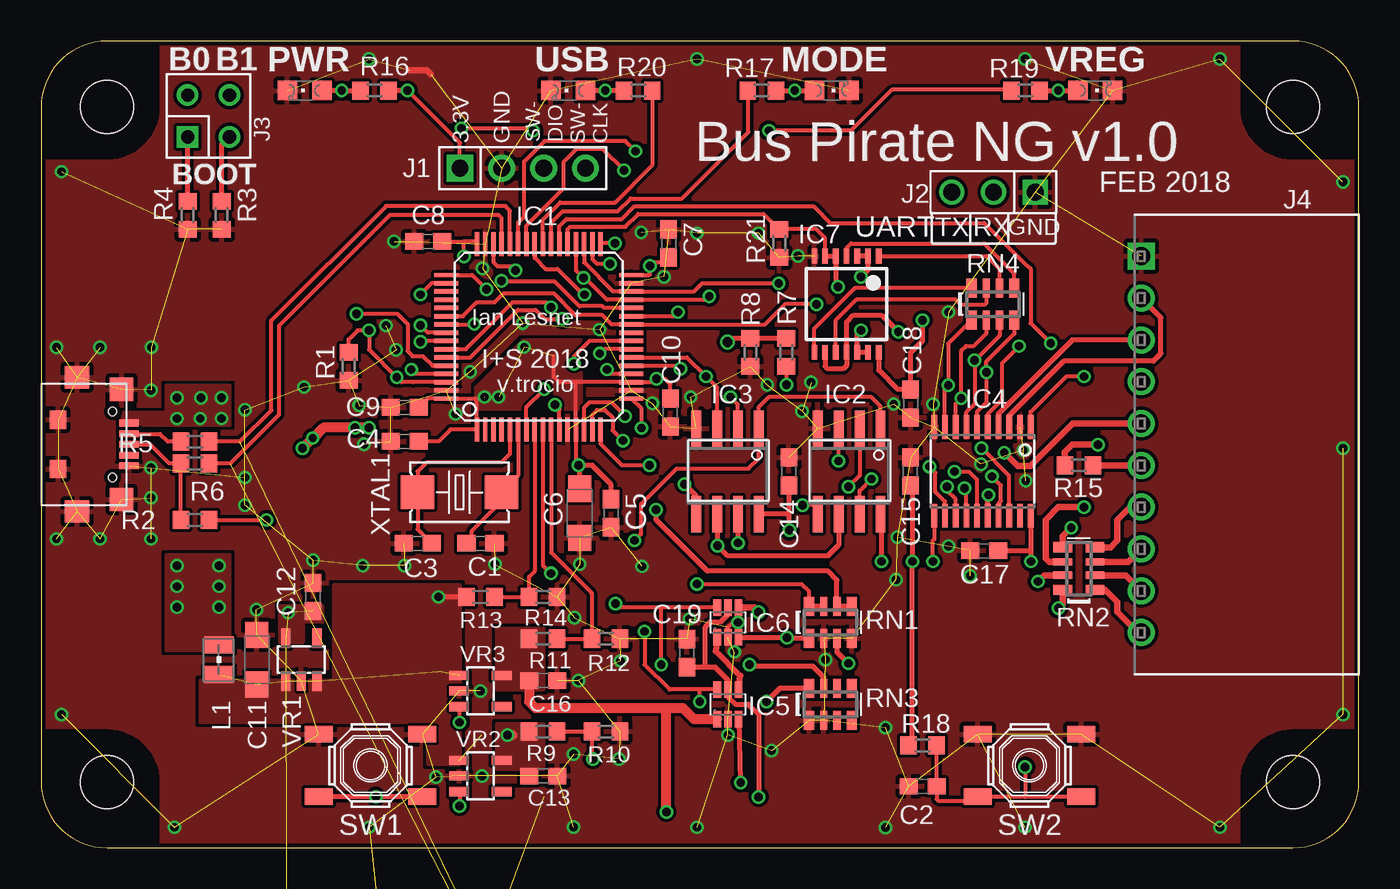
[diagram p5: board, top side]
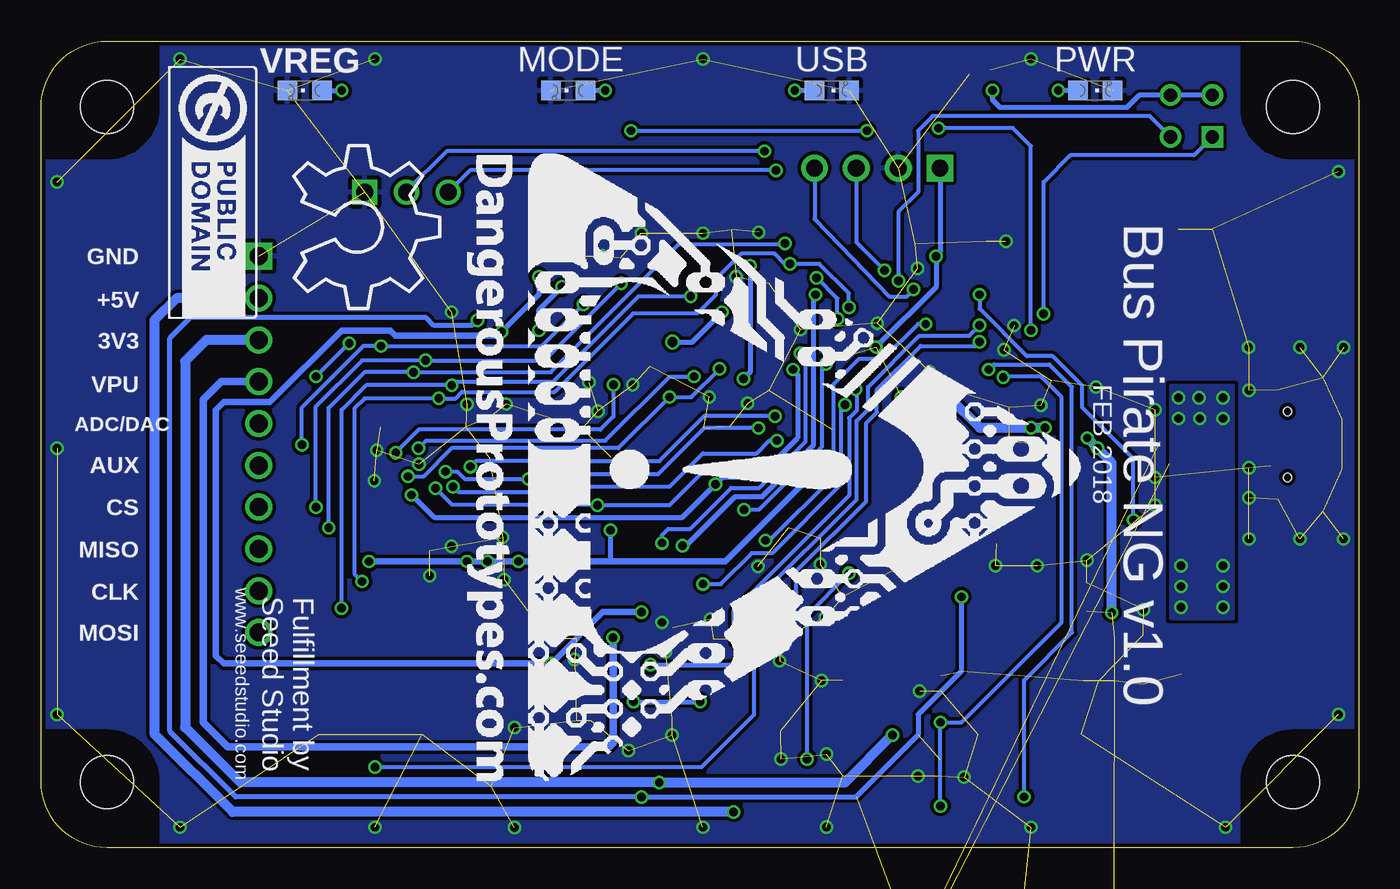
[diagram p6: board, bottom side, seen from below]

Size 80 x 49 mm. Coordinates in mm from the lower left corner, seen from the top.
Copper layers (1*16): Top 0.035mm / dielectric 1.5mm / Bottom 0.035mm
Design rules "dirt_cheap_dirty_boards.v1.1": minimum track width 6mil, minimum drill 12mil, track to track 6mil, track to pad 6mil, pad to pad 6mil, via to via 6mil, smd to smd 0mil, copper to edge 10mil, drill to drill 10mil, minimum pad ring 10mil, minimum via ring 6mil, stop-mask expansion 2mil, vias tented up to drill 25mil, thermal gap 10mil

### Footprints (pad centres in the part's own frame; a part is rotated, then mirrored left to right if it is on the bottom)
C0603 = smd 1.1 x 1: 1 -0.85,0; 2 0.85,0
SMC_A = smd 1.6 x 1.4: + -1.5,0; - 1.5,0
CON_USB_MICRO-B-1-MD05SMXXX-01 = smd 1.35 x 1.5: GND1 -4.075,0; GND2 4.075,0 | smd 1.4 x 1.4: GND3 -3.35,2.7; GND4 3.35,2.7 | smd 1.1 x 1: GND5 -1.5,-1.15; GND6 1.5,-1.15 | smd 0.4 x 1.2: P1 -1.3,3.16; P2 -0.65,3.16; P3 0,3.16; P4 0.65,3.16; P5 1.3,3.16 | hole 0.5: -2,2.15; 2,2.15
LQFP64 = smd 1.45 x 0.27: 1 -5.625,3.75; 2 -5.625,3.25; 3 -5.625,2.75; 4 -5.625,2.25; 5 -5.625,1.75; 6 -5.625,1.25; 7 -5.625,0.75; 8 -5.625,0.25; 9 -5.625,-0.25; 10 -5.625,-0.75; 11 -5.625,-1.25; 12 -5.625,-1.75; 13 -5.625,-2.25; 14 -5.625,-2.75; 15 -5.625,-3.25; 16 -5.625,-3.75; 33 5.625,-3.75; 34 5.625,-3.25; 35 5.625,-2.75; 36 5.625,-2.25; 37 5.625,-1.75; 38 5.625,-1.25; 39 5.625,-0.75; 40 5.625,-0.25; 41 5.625,0.25; 42 5.625,0.75; 43 5.625,1.25; 44 5.625,1.75; 45 5.625,2.25; 46 5.625,2.75; 47 5.625,3.25; 48 5.625,3.75 | smd 0.27 x 1.45: 17 -3.75,-5.625; 18 -3.25,-5.625; 19 -2.75,-5.625; 20 -2.25,-5.625; 21 -1.75,-5.625; 22 -1.25,-5.625; 23 -0.75,-5.625; 24 -0.25,-5.625; 25 0.25,-5.625; 26 0.75,-5.625; 27 1.25,-5.625; 28 1.75,-5.625; 29 2.25,-5.625; 30 2.75,-5.625; 31 3.25,-5.625; 32 3.75,-5.625; 49 3.75,5.625; 50 3.25,5.625; 51 2.75,5.625; 52 2.25,5.625; 53 1.75,5.625; 54 1.25,5.625; 55 0.75,5.625; 56 0.25,5.625; 57 -0.25,5.625; 58 -0.75,5.625; 59 -1.25,5.625; 60 -1.75,5.625; 61 -2.25,5.625; 62 -2.75,5.625; 63 -3.25,5.625; 64 -3.75,5.625
SOIC-8 = smd 0.6 x 2.2: 1 -1.905,-2.6; 2 -0.635,-2.6; 3 0.635,-2.6; 4 1.905,-2.6; 5 1.905,2.6; 6 0.635,2.6; 7 -0.635,2.6; 8 -1.905,2.6
TSSOP-20 = smd 0.35 x 1.43: 1 -2.925,-2.7; 2 -2.275,-2.7; 3 -1.625,-2.7; 4 -0.975,-2.7; 5 -0.325,-2.7; 6 0.325,-2.7; 7 0.975,-2.7; 8 1.625,-2.7; 9 2.275,-2.7; 10 2.925,-2.7; 11 2.925,2.7; 12 2.275,2.7; 13 1.625,2.7; 14 0.975,2.7; 15 0.325,2.7; 16 -0.325,2.7; 17 -0.975,2.7; 18 -1.625,2.7; 19 -2.275,2.7; 20 -2.925,2.7
SC-70-6 = smd 0.47 x 1: 1 -0.65,-0.9; 2 0,-0.9; 3 0.65,-0.9; 4 0.65,0.9; 5 0,0.9; 6 -0.65,0.9
40XX_TSSOP14 = smd 0.35 x 0.9: 1 -1.95,-2.925; 2 -1.3,-2.925; 3 -0.65,-2.925; 4 0,-2.925; 5 0.65,-2.925; 6 1.3,-2.925; 7 1.95,-2.925; 8 1.95,2.925; 9 1.3,2.925; 10 0.65,2.925; 11 0,2.925; 12 -0.65,2.925; 13 -1.3,2.925; 14 -1.95,2.925
SOT23-5 = smd 0.69 x 0.99: 1 -0.95,-1.29; 2 0,-1.29; 3 0.95,-1.29; 4 0.95,1.3; 5 -0.95,1.3
DBV-R-PDSO-G6 = smd 0.69 x 0.99: 1 -0.95,-1.29; 2 0,-1.29; 3 0.95,-1.29; 4 0.95,1.3; 5 0,1.3; 6 -0.95,1.3
M1X4 = drill 1.02 pad 1.632 square: 1 0,0 | drill 1.02 pad 1.632: 2 2.54,0; 3 5.08,0; 4 7.62,0
M1X3 = drill 1.02 square: 1 0,0 | drill 1.02: 2 2.54,0; 3 5.08,0
M2X2 = drill 0.8 square: 1 -1.27,-1.27 | drill 0.8: 2 -1.27,1.27; 3 1.27,-1.27; 4 1.27,1.27
M1X10_MALE_RIGHT_ANGLES_PTH_SHROUDED = drill 1.09 square: 1 -11.43,-6.415 | drill 1.09: 2 -8.89,-6.415; 3 -6.35,-6.415; 4 -3.81,-6.415; 5 -1.27,-6.415; 6 1.27,-6.415; 7 3.81,-6.415; 8 6.35,-6.415; 9 8.89,-6.415; 10 11.43,-6.415
WE-KI_0805_B = smd 1.02 x 1.78: 1 -0.89,0; 2 0.89,0
LED-805 = smd 1.2 x 1.2: A 0,-1.05; C 0,1.05
DP8049_V1 = hole 3.2: -36,-20.5; 36,-20.5; 36,20.5; -36,20.5
R603 = smd 1 x 1.1: 1 -0.85,0; 2 0.85,0
R0603 = smd 1 x 1.1: 1 -0.85,0; 2 0.85,0
RN8P-4R-CRA06S = smd 0.63 x 1.15: 1 -1.295,-0.975; 4 1.295,-0.975; 5 1.295,0.975; 8 -1.295,0.975 | smd 0.44 x 1.15: 2 -0.4,-0.975; 3 0.4,-0.975; 6 0.4,0.975; 7 -0.4,0.975
SW_TACT_SMALL = smd 1.7 x 1: 1 -3.15,1.9; 2 3.15,1.9; 3 -3.15,-1.9; 4 3.15,-1.9
TQFP-144 = smd 0.9 x 0.3: 1 -10.75,8.75; 2 -10.75,8.25; 3 -10.75,7.75; 4 -10.75,7.25; 5 -10.75,6.75; 6 -10.75,6.25; 7 -10.75,5.75; 8 -10.75,5.25; 9 -10.75,4.75; 10 -10.75,4.25; 11 -10.75,3.75; 12 -10.75,3.25; 13 -10.75,2.75; 14 -10.75,2.25; 15 -10.75,1.75; 16 -10.75,1.25; 17 -10.75,0.75; 18 -10.75,0.25; 19 -10.75,-0.25; 20 -10.75,-0.75; 21 -10.75,-1.25; 22 -10.75,-1.75; 23 -10.75,-2.25; 24 -10.75,-2.75; 25 -10.75,-3.25; 26 -10.75,-3.75; 27 -10.75,-4.25; 28 -10.75,-4.75; 29 -10.75,-5.25; 30 -10.75,-5.75; 31 -10.75,-6.25; 32 -10.75,-6.75; 33 -10.75,-7.25; 34 -10.75,-7.75; 35 -10.75,-8.25; 36 -10.75,-8.75; 73 10.75,-8.75; 74 10.75,-8.25; 75 10.75,-7.75; 76 10.75,-7.25; 77 10.75,-6.75; 78 10.75,-6.25; 79 10.75,-5.75; 80 10.75,-5.25; 81 10.75,-4.75; 82 10.75,-4.25; 83 10.75,-3.75; 84 10.75,-3.25; 85 10.75,-2.75; 86 10.75,-2.25; 87 10.75,-1.75; 88 10.75,-1.25; 89 10.75,-0.75; 90 10.75,-0.25; 91 10.75,0.25; 92 10.75,0.75; 93 10.75,1.25; 94 10.75,1.75; 95 10.75,2.25; 96 10.75,2.75; 97 10.75,3.25; 98 10.75,3.75; 99 10.75,4.25; 100 10.75,4.75; 101 10.75,5.25; 102 10.75,5.75; 103 10.75,6.25; 104 10.75,6.75; 105 10.75,7.25; 106 10.75,7.75; 107 10.75,8.25; 108 10.75,8.75 | smd 0.3 x 0.9: 37 -8.75,-10.75; 38 -8.25,-10.75; 39 -7.75,-10.75; 40 -7.25,-10.75; 41 -6.75,-10.75; 42 -6.25,-10.75; 43 -5.75,-10.75; 44 -5.25,-10.75; 45 -4.75,-10.75; 46 -4.25,-10.75; 47 -3.75,-10.75; 48 -3.25,-10.75; 49 -2.75,-10.75; 50 -2.25,-10.75; 51 -1.75,-10.75; 52 -1.25,-10.75; 53 -0.75,-10.75; 54 -0.25,-10.75; 55 0.25,-10.75; 56 0.75,-10.75; 57 1.25,-10.75; 58 1.75,-10.75; 59 2.25,-10.75; 60 2.75,-10.75; 61 3.25,-10.75; 62 3.75,-10.75; 63 4.25,-10.75; 64 4.75,-10.75; 65 5.25,-10.75; 66 5.75,-10.75; 67 6.25,-10.75; 68 6.75,-10.75; 69 7.25,-10.75; 70 7.75,-10.75; 71 8.25,-10.75; 72 8.75,-10.75; 109 8.75,10.75; 110 8.25,10.75; 111 7.75,10.75; 112 7.25,10.75; 113 6.75,10.75; 114 6.25,10.75; 115 5.75,10.75; 116 5.25,10.75; 117 4.75,10.75; 118 4.25,10.75; 119 3.75,10.75; 120 3.25,10.75; 121 2.75,10.75; 122 2.25,10.75; 123 1.75,10.75; 124 1.25,10.75; 125 0.75,10.75; 126 0.25,10.75; 127 -0.25,10.75; 128 -0.75,10.75; 129 -1.25,10.75; 130 -1.75,10.75; 131 -2.25,10.75; 132 -2.75,10.75; 133 -3.25,10.75; 134 -3.75,10.75; 135 -4.25,10.75; 136 -4.75,10.75; 137 -5.25,10.75; 138 -5.75,10.75; 139 -6.25,10.75; 140 -6.75,10.75; 141 -7.25,10.75; 142 -7.75,10.75; 143 -8.25,10.75; 144 -8.75,10.75
SOT-23-5@1 = smd 0.55 x 1.2: 1 -0.95,-1.3; 2 0,-1.3; 3 0.95,-1.3; 4 0.95,1.3; 5 -0.95,1.3
XTAL_4X6 = smd 2.032 x 2.032: 1 -2.54,0; 2 2.54,0

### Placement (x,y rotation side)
C1  26.67,18.49 180 top
C2  53.52,3.73 0 top
C3  22.86,18.49 0 top
C4  22.07,24.69 0 top
C5  34.61,20.32 90 top
C6  32.7,20.32 270 top
C7  38.1,36.72 270 top
C8  23.5,36.83 0 top
C9  22.07,26.75 0 top
C10  38.21,26.44 90 top
C11  13.1,11.43 90 top
C12  16.51,15.24 90 top
C13  30.48,4.37 0 top
C14  45.4,22.86 90 top
C15  52.78,22.86 90 top
C16  30.48,10.16 0 top
C17  57.25,18.05 180 top
C18  52.78,26.99 270 top
C19  39.2,11.82 90 top
C20  not placed on the board
C21  not placed on the board
C22  not placed on the board
C23  not placed on the board
C24  not placed on the board
C25  not placed on the board
C26  not placed on the board
C27  not placed on the board
C28  not placed on the board
C29  not placed on the board
C30  not placed on the board
C31  not placed on the board
C32  not placed on the board
C33  not placed on the board
C34  not placed on the board
C35  not placed on the board
C36  not placed on the board
C37  not placed on the board
C38  not placed on the board
C39  not placed on the board
C40  not placed on the board
C41  not placed on the board
C42  not placed on the board
C43  not placed on the board
CON1  2.18,24.5 270 top
IC1  30.21,31.04 90 top
IC2  49.05,22.86 180 top
IC3  41.67,22.86 180 top
IC4  57.15,22.86 180 top
IC5  41.69,8.71 0 top
IC6  41.69,13.69 0 top
IC7  48.9,33.02 180 top
IC8  not placed on the board
IC9  not placed on the board
IC10  not placed on the board
IC11  not placed on the board
IC12  not placed on the board
IC13  not placed on the board
IC14  not placed on the board
IC15  not placed on the board
IC16  not placed on the board
IC17  not placed on the board
J1  25.43,41.29 0 top
J2  60.36,39.83 180 top
J3  10.16,44.45 0 top
J4  73.2,24.5 270 top
L1  10.79,11.43 90 top
LED1  16,46 270 bottom
LED2  16,46 90 top
LED3  48,46 270 top
LED4  48,46 90 bottom
LED5  64,46 270 top
LED6  64,46 90 bottom
LED7  32,46 90 top
LED8  32,46 270 bottom
LOGO1  72.27,47.47 270 bottom
PCB1  40,24.5 0 top
R1  18.67,29.25 270 top
R2  9.33,19.91 0 top
R3  10.95,38.43 270 top
R4  8.89,38.43 270 top
R5  9.34,24.67 180 top
R6  9.33,23.35 180 top
R7  45.24,30.09 90 top
R8  43.06,30.09 90 top
R9  30.48,7.06 0 top
R10  34.29,7.06 180 top
R11  30.48,12.7 0 top
R12  34.29,12.7 180 top
R13  26.67,15.24 0 top
R14  30.48,15.24 180 top
R15  63,23.23 0 top
R16  20.25,46 0 top
R17  43.75,46 180 top
R18  53.52,6.22 180 top
R19  59.75,46 180 top
R20  36.25,46 0 top
R21  44.81,36.72 270 top
R22  not placed on the board
R23  not placed on the board
R24  not placed on the board
R25  not placed on the board
R26  not placed on the board
R27  not placed on the board
R28  not placed on the board
R29  not placed on the board
R30  not placed on the board
R31  not placed on the board
R32  not placed on the board
R33  not placed on the board
R34  not placed on the board
R35  not placed on the board
R36  not placed on the board
R37  not placed on the board
R38  not placed on the board
R39  not placed on the board
RN1  47.92,13.69 0 top
RN2  63.01,16.96 90 top
RN3  47.92,8.71 0 top
RN4  57.78,33.02 0 top
SW1  20,5 180 top
SW2  60,5 180 top
U1  not placed on the board
U2  not placed on the board
U3  not placed on the board
U$1  [DP-LOGO]  not placed on the board
U$2  [OSHW_8X350_NOTEXT]  64.67,42.67 270 bottom
U$4  [DP_LOGO_ART_1.5X1.5]  54.12,42.15 270 bottom
VR1  15.8,11.43 0 top
VR2  26.67,4.37 270 top
VR3  26.67,9.53 270 top
VR4  not placed on the board
XTAL1  25.4,21.59 180 top
XTAL2  not placed on the board

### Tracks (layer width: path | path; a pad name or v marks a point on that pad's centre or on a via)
1V2  (7 unrouted)
3V3  (via drill 0.51)  (43 unrouted)
  Top 0.254: C8.2 25.67,36.83 | C4.2 24.13,24.69 24.86,25.41 IC1.1 26.46,27.26 26.43,27.29 IC1.64 23.46,27.29 C9.2 | C7.2 38.1,35.56 37.17,35.56 v36.96,35.35 36.96,34.85 36.91,34.79 IC1.32 35.77,34.79 | 32.46,28.29 IC1.19 37.14,28.29 v37.35,28.5 37.85,28.5 38.21,28.14 C10.2 | 32.46,28.29 IC1.13 32.46,23.4 | IC4.11 54.23,18.75 54.14,18.67 v54.14,17.4 | 32.46,28.29 31.45,28.29 31.11,28.63 31.11,29.87 | v25.67,35.94 25.67,36.83 | IC1.48 26.46,36.83 25.67,36.83 | 52.9,6.45 R18.2 | J1.1 25.43,42.83 v22.25,46
  Top 0.305: v22.25,46 R16.2 | 51.02,20.32 IC2.8 51.03,20.19 v51.03,17.4 | IC3.8 43.64,20.32 45.37,20.32 45.43,20.38 | IC4.20 60.08,20.31 60.09,20.32 60.09,18.05 | 60.09,18.05 v60.09,17.4 | 32.46,23.4 v32.62,23.24 | C5.2 34.61,22.07 33.43,23.24 v32.62,23.24 | C6.+ 32.7,23.16 v32.62,23.24 | IC4.11 54.23,20.32 | C15.1 52.9,21.9 v52.9,17.4 52.9,6.45 | C17.1 60.09,18.05 | v45.43,19.29 45.43,20.38 | 45.43,20.38 45.43,21.98 C14.1
  Top 0.61: v19.91,25.51 17.13,25.51 16.51,24.89 v16.49,24.89 v15.87,24.27
  Bottom 0.305: 46.67,17.4 49.76,17.4 49.78,17.42 45.43,17.42 v45.43,19.29 | J3.2 J3.4 13.32,45.72 14.08,44.96 21.78,44.96 22.25,45.43 v22.25,46 | v36.96,35.35 36.96,28.89 v37.35,28.5 | v29.33,30.41 25.67,34.07 v25.67,35.94 25.43,36.18 J1.1
  Bottom 0.406: v32.62,23.24 38.47,17.4 46.67,17.4 v51.03,17.4 v52.9,17.4 v54.14,17.4 v60.09,17.4
  Bottom 0.61: 16.51,24.87 v16.49,24.89 v15.87,24.27 15,23.4 v15,14.29 | v19.06,25.51 v19.91,25.51 23.02,25.51 24.89,27.38 v26.91,27.38 v26.92,27.38 v27.77,27.38
  pour Top (isolate 0.152, no thermals): 29.29,30.84 32.76,30.84 32.76,26.65 26.41,26.65 26.41,27.97
  pour Top (no thermals): 14.53,14.68 17.07,14.68 17.07,13.73 15.88,13.73 15.88,12.46 14.53,12.46
+3V3  (1 unrouted)
ADC1  (via drill 0.51, 0.58)
  Top 0.254: IC1.27 38.4,32.29 v38.66,32.54
  Top 0.305: 41.63,30.68 v41.67,30.72 41.9,30.94 R8.2 R7.2
  Bottom 0.305: v41.67,30.72 40.48,30.72 v38.66,32.54
ADC2  (via drill 0.51)
  Top 0.254: v39.83,16.02 46.16,16.02 46.62,15.56 RN1.8 | IC1.11 31.46,26.65 v31.2,26.91
  Top 0.305: RN1.7 RN1.8
  Bottom 0.254: v39.83,16.02 38.74,16.02 36.87,17.89 35.63,17.89 31.43,22.09 31.43,26.67 v31.2,26.91
ADC3  (via drill 0.51)
  Top 0.254: R9.2 R10.2 33.44,5.45 v33.5,5.4 | IC1.9 30.46,17.16 v30.96,16.67
  Bottom 0.254: v33.5,5.4 33.5,14.13 v30.96,16.67
ADC4
  Top 0.254: R11.2 R12.2 33.42,12.72 33.42,15.48 30.96,17.93 IC1.10
ADC5
  Top 0.254: R13.2 R14.2 29.63,16.45 29.96,16.78 IC1.8
ADC6  (via drill 0.51)
  Top 0.254: IC1.24 33.28,30.79 32.36,29.87 v32.36,29.4
  Top 0.305: v37.34,20.54 37.34,19.91 40.45,16.8 47.76,16.8 48.32,16.25 RN1.6 RN1.5
  Bottom 0.254: v37.34,20.54 36.41,20.54 32.59,24.35 32.59,29.17 v32.36,29.4
AUX0  (via drill 0.51)
  Top 0.254: v47.07,33.02 45.16,33.02 43.93,31.79 IC1.26 34.64,31.79 34.07,32.36 32.44,32.36 31.11,33.68 28.08,33.68 27.54,33.14 26.45,33.14 25.6,32.29 IC1.54 | IC4.5 57.48,26.36 58.34,27.23 58.34,29.44 v59.38,30.48
  Top 0.406: v64.17,24.48 62.6,24.48 62.15,24.04 R15.1
  Bottom 0.254: v47.07,33.02 49.61,30.48 v59.38,30.48 60.44,30.48 64.17,26.75 v64.17,24.48
BOOT0  (via drill 0.51)
  Top 0.254: IC1.60 23.76,29.29 23.18,29.87 22.56,29.87 22.25,30.18 22.25,31.82 21.62,32.44 v19.14,32.44
  Top 0.305: R4.1 J3.1
  Bottom 0.254: J3.1 10,42.07 17.52,42.07 19.14,40.45 v19.14,32.44
BOOT1  (via drill 0.51)
  Top 0.254: IC1.28 34.19,32.79 34.07,32.9 32.67,32.9 31.19,34.38 28,34.38 v27.94,34.44
  Top 0.305: R3.1 10.95,42.7 J3.3
  Bottom 0.254: J3.3 12.7,44.45 25.87,44.45 26.76,43.56 26.76,39.83 27.93,38.66 27.93,34.46 v27.94,34.44
BPIO_AUX  (2 unrouted)
BPIO_CLOCK  (2 unrouted)
BPIO_CS  (2 unrouted)
BPIO_MISO  (2 unrouted)
BPIO_MOSI  (2 unrouted)
BUFDIR_AUX  (1 unrouted)
BUFDIR_CLOCK  (1 unrouted)
BUFDIR_CS  (1 unrouted)
BUFDIR_MISO  (1 unrouted)
BUFDIR_MOSI  (1 unrouted)
BUFOD_AUX  (1 unrouted)
BUFOD_CLOCK  (1 unrouted)
BUFOD_CS  (1 unrouted)
BUFOD_MISO  (1 unrouted)
BUFOD_MOSI  (1 unrouted)
CLOCK  (via drill 0.51)
  Top 0.254: IC4.8 55.52,26.97 v55.86,27.3 55.86,30.19 56.16,30.49 56.63,30.49 57.38,31.25 RN4.2 | IC1.58 25.78,30.29 28.63,33.14 30.65,33.14 v30.96,32.83 | v34.54,35.47 33.76,35.47 33.46,35.77 IC1.34
  Top 0.406: RN2.7 60.9,16.56 v60.52,16.18
  Bottom 0.254: v60.52,16.18 60.98,16.65 60.98,26.68 60.36,27.3 v55.86,27.3 54.84,27.3 54.45,27.69 48.83,27.69 44.06,32.46 40.16,32.46 39.05,33.58 39.05,34.54 37.49,36.09 35.47,36.09 34.85,35.47 v34.54,35.47 32.75,35.47 30.96,33.68 v30.96,32.83
CS  (via drill 0.51)
  Top 0.254: IC4.6 56.83,26.49 57.39,27.05 v57.39,28.89 57.39,29.54 59.08,31.23 RN4.4 | v34.84,36.72 34.02,36.72 IC1.33
  Top 0.406: RN2.5 62.03,18.94 v62.54,19.45
  Bottom 0.254: v62.54,19.45 62.54,26.71 60.36,28.89 v57.39,28.89 49.06,28.89 41.31,36.64 34.93,36.64 v34.84,36.72
D+
  Top 0.254: CON1.P3 6.62,24.5 7.76,23.35 R6.2 R2.1
D-
  Top 0.254: CON1.P2 7.21,25.15 7.69,24.67 R5.2
EXVUSB  (via drill 0.51)
  other vias: 9.71,27.34 10.95,27.34 10.95,26.07 8.26,26.07 8.26,27.34 9.66,26.07 10.79,17.14 8.26,17.14 8.26,15.88 10.79,15.88 10.79,14.61 8.26,14.61
  pour Top (isolate 0.305, no thermals): 4.99,26.43 7.62,26.43 7.62,28.09 11.43,28.09 11.43,25.68 4.99,25.68
  pour Top (no thermals): 7.62,17.78 11.43,17.78 11.43,11.99 7.62,11.99
  pour Bottom: 7.62,28.04 11.43,28.04 11.43,13.97 7.62,13.97
FLASH_MISO  (1 unrouted)
FLASH_MOSI  (1 unrouted)
FLASH_SCK  (1 unrouted)
FPGA_PROG_CS  (1 unrouted)
GND  (via drill 0.51)  (217 unrouted)
  Top 0.254: 41.69,12.76 41.69,13.38 42.01,13.69 v42.32,13.69
  Top 0.406: 22.38,47.23 23.42,47.23 23.65,46.99
  other vias: 19.6,24.52 44.08,28.12 71.56,47.92 19.91,47.92 32.33,5.68 55.09,32.54 19.91,1.24 26.05,28.91 39.83,1.24 45.96,35.96 0.93,18.76 39.83,37.34 42.08,11.9 79.03,40.45 12.37,20.81 36.49,17.09 39.44,27.38 16.51,17.46 22.07,17.14 19.31,26.88 23.97,4.29 59.74,47.92 79.03,24.27 8.09,1.24 6.68,23.09 12.37,26.61 6.68,18.76 79.03,8.09 43.56,37.34 37.8,34.69 32.62,10.16 39.83,47.92 35.16,11.35 21.43,36.83 13.07,14.47 71.56,1.24 1.24,41.07 32.7,17.22 35.08,5.4 1.24,8.09 51.27,7.3 6.68,21.26 59.74,1.24 46.74,28.27 46.2,26.52 36.43,37.39 19.53,17.14 15.95,27.99 27.54,17.22 3.58,18.76 25.16,26.35 12.37,22.49 32.38,13.97 26.67,9.53 26.76,4.36 56.41,16.52 59.62,24.16 6.69,30.4 6.68,27.79 0.93,30.4 41.69,6.85 59.78,22.29 3.58,30.4 54.16,26.94 44.35,5.9 51.27,1.23 32.33,1.25 57.06,23.3 51.77,26.96 55.09,18.31 51.98,18.86 51.9,16.29 47.61,11.42 39.37,13.9 26.8,35.2 29.24,31.87 33.91,31.48 37.1,26.99 20.93,31.72 21.55,30.24
  pour Top (isolate 0.203, rank 2): 0,48.97 80.01,48.97 80.01,0 0,0
  pour Bottom (isolate 0.203, rank 2): 0,48.97 80.01,48.97 arc-3 80.01,0 0,0
IO_ADC/DAC  (via drill 0.51)
  Top 0.254: v45.26,28.13 45.26,29.22 R7.1
  Top 0.406: J4.5 62.64,25.77 60.05,23.18 59.29,23.18 v58.47,24
  Bottom 0.254: v58.47,24 57.07,25.4 46.05,25.4 45.26,26.19 v45.26,28.13
IO_AUX0
  Top 0.406: J4.6 R15.2
IO_CLK
  Top 0.406: RN2.2 65.84,16.56 J4.9
IO_CS
  Top 0.406: RN2.4 64.92,18.25 65.34,18.67 65.34,19.91 66.12,20.69 J4.7
IO_MISO
  Top 0.406: RN2.3 66,17.36 J4.8
IO_MOSI
  Top 0.406: RN2.1 64.61,15.66 65.34,14.94 65.34,14.31 66.58,13.07 J4.10
IO_OE  (via drill 0.51)
  Top 0.254: v61.3,30.65 60.08,31.87 60.08,35.17 59.74,35.47 57.25,37.96 47.92,37.96 46.91,38.97 36.02,38.97 35.24,38.19 31.89,38.19 31.46,37.76 IC1.38 | v63.32,28.63 62.23,28.63 60.08,26.47 IC4.1
  Bottom 0.254: v61.3,30.65 v63.32,28.63
LA_AUX0  (via drill 0.51)
  Top 0.254: IC1.20 34.61,28.79 v34.35,29.05
  Top 0.305: IC4.16 57.48,21.39 v57.51,21.43 | IC3.5 39.77,21.37 v39.05,22.09
  Bottom 0.305: v34.35,29.05 34.07,28.77 34.07,24.89 36.48,22.48 38.66,22.48 v39.05,22.09 41.07,20.07 56.15,20.07 v57.51,21.43
LA_CLK  (via drill 0.51)
  Top 0.254: IC2.2 49.69,22.62 v49.01,21.94 | IC4.13 55.52,21.17 55,21.7 v55,21.94 | IC1.15 33.46,26.3 33.76,26.6 34.23,26.6 34.69,26.14 34.69,25.36 v35.32,24.74
  Bottom 0.254: v55,21.94 54.69,21.62 49.32,21.62 v49.01,21.94 41.85,21.94 39.83,23.96 36.56,23.96 35.78,24.74 v35.32,24.74
LA_CS  (via drill 0.51)
  Top 0.254: 49.69,20.64 IC2.7 49.69,21.68 v50.41,22.4 | IC4.15 56.83,22.33 56.3,22.85 v55.45,22.85 | v36.45,25.5 36.45,26.68 IC1.17
  Top 0.305: 49.69,20.16 IC2.7
  Bottom 0.254: v36.45,25.5 39.74,25.5 42.55,22.7 50.11,22.7 v50.41,22.4 54.3,22.4 54.75,22.85 v55.45,22.85
LA_HOLD  (via drill 0.51)
  Top 0.254: IC1.23 34.18,30.29 v33.91,30.03
  Top 0.305: IC3.7 42.31,18.52 v42.32,18.51
  Bottom 0.254: v33.91,30.03 33.6,29.71 33.6,24.66 36.41,21.86 38.12,21.86 40.6,19.37 41.93,19.37 42.32,18.98 v42.32,18.51
LA_MISO  (via drill 0.51)
  Top 0.254: IC1.16 33.97,24.53 35.27,23.23 v36.94,23.23 | IC4.14 56.17,21.71 v56.05,21.83 | IC2.5 47.15,20.69 47.29,20.83 46.24,20.83 v46.23,20.82
  Bottom 0.254: v56.05,21.83 55.07,20.85 48.22,20.85 v46.23,20.82 41.85,20.82 39.43,23.23 v36.94,23.23
LA_MOSI  (via drill 0.51)
  Top 0.254: v48.42,23.5 IC2.3 | IC4.12 54.88,21.05 54.3,21.62 54.3,22.79 v53.92,23.16 | IC1.14 32.96,26.74 33.29,27.07 34.6,27.07 v35.45,26.22
  Bottom 0.254: v35.45,26.22 39.74,26.22 42.47,23.5 v48.42,23.5 53.59,23.5 v53.92,23.16
LA_SWV33  (via drill 0.51)
  Top 0.254: IC1.21 38.62,29.29 v38.82,29.09 | v57.72,22.56 58.26,22.01 58.26,21.08 58.12,20.94 IC4.17 | IC3.2 42.31,26.92 v41.85,27.38
  Bottom 0.254: v38.82,29.09 40.53,27.38 v41.85,27.38 44.96,24.27 55.07,24.27 56.78,22.56 v57.72,22.56
LA_SWV50  (via drill 0.51)
  Top 0.254: IC1.22 39.21,29.79 v40.37,28.63 41.04,27.96 IC3.3 | IC4.18 58.77,22.59 v57.1,24.27
  Bottom 0.254: v40.37,28.63 41.85,28.63 45.74,24.74 56.63,24.74 v57.1,24.27
LD1
  Top 0.254: IC1.39 30.96,37.96 31.66,38.66 35,38.66 35.78,39.44 38.89,39.44 42.94,43.48 42.94,45.96 R17.2
MISO  (via drill 0.51)
  Top 0.254: IC4.7 56.17,26.46 56.67,26.96 v56.67,29.61 58.19,31.12 RN4.3 | v44.78,34.28 40.11,34.28 39.62,33.79 IC1.30 34.74,33.79 32.96,35.57 IC1.35
  Top 0.406: v63.32,20.69 61.76,20.69 60.98,19.91 60.98,17.58 61.21,17.36 RN2.6
  Bottom 0.254: v44.78,34.28 49.45,29.61 v56.67,29.61 60.52,29.61 63.32,26.81 v63.32,20.69
MOSI  (via drill 0.51)
  Top 0.254: IC1.36 32.46,35.09 v32.92,34.63 33,34.63 34.34,33.29 IC1.29 40.29,33.29 40.5,33.5 v40.56,33.5 | RN4.1 55.07,30.62 v55.07,28.1 54.88,27.9 IC4.9 | IC1.59 26.06,29.79 28.94,32.67 30.03,32.67 30.57,32.13 v31.66,32.13
  Top 0.406: RN2.8 62.03,14.82 v61.76,14.55
  Bottom 0.254: v40.56,33.5 43.74,33.5 48.92,28.32 54.76,28.32 54.98,28.1 v55.07,28.1 60.27,28.1 61.76,26.6 v61.76,14.55 | v31.66,32.13 31.66,33.37 v32.92,34.63
MS0  (via drill 0.51)
  Top 0.254: IC1.61 22.73,28.79 v22.47,29.05
  Top 0.305: SW1.2 17.46,3.1 v20.32,3.1 22.54,3.1 SW1.1
  Bottom 0.254: v22.47,29.05 22.16,29.37 18.79,29.37 17.42,28 17.42,13.07 20.32,10.17 v20.32,3.1
N$1
  Top 0.356: IC6.1 40.94,11.95 42.44,10.45 IC5.4
N$2
  Top 0.254: IC7.1 57.4,35.95 58.19,35.16 RN4.6
N$3
  Top 0.254: IC7.4 48.9,36.45 49.16,36.72 57.25,36.72 59.08,34.89 RN4.5
N$4
  Top 0.254: RN4.8 49.4,33.99 46.95,31.54 IC7.8
N$5
  Top 0.254: RN4.7 57.38,33.12 57.25,32.98 55.85,32.98 55.54,33.29 49.47,33.29 48.24,32.06 IC7.10
N$6  (via drill 0.51)
  Top 0.305: R17.1 v45.75,46 LED4.A
  Bottom 0.305: v45.75,46 LED4.A
N$7  (via drill 0.51)
  Top 0.305: R16.1 v18.25,46 LED1.A
  Bottom 0.305: LED1.A v18.25,46
N$8  (2 unrouted)
N$9  (2 unrouted)
N$12  (1 unrouted)
N$13  (via drill 0.51)
  Top 0.305: LED8.A v34.25,46 R20.1
  Bottom 0.305: LED8.A v34.25,46
N$14  (1 unrouted)
N$16
  Top 0.254: IC1.5 28.46,23.94 27.94,23.42 23.42,23.42 22.86,22.86 XTAL1.2 22.86,19.34 C3.2
N$18  (via drill 0.51)
  Top 0.305: R19.1 v61.75,46 LED6.A
  Bottom 0.305: LED6.A v61.75,46
N$20
  Top 0.254: IC1.6 28.96,22.61 XTAL1.1 27.94,21.03 26.11,19.21 26.11,18.79 C1.2
RST  (via drill 0.51)
  Top 0.254: IC1.7 29.46,26.76 v30.54,27.84 | 57.46,3.1 59.74,3.1 | 62.54,3.1 59.74,3.1 | v59.74,4.91 59.74,3.1 | R18.1 C2.2 54.37,2.95 54.46,2.86 56.61,2.86 SW2.2
  Top 0.305: SW2.1 62.54,3.1 | SW2.2 57.46,3.1
  Bottom 0.254: v59.74,4.91 39.9,4.91 36.72,8.09 36.72,11.2 37.96,12.45 37.96,14.39 30.95,21.4 30.95,26.12 30.47,26.6 30.47,27.77 v30.54,27.84
SRAM_CLK  (via drill 0.51)
  Top 0.254: IC1.41 29.96,35.85 30.65,35.16 31.35,35.16 32.9,33.6 v32.98,33.6
  Top 0.305: IC2.6 48.42,18.39 47.76,17.74 41.69,17.74 v41.07,18.36 41.04,18.39 IC3.6
  Bottom 0.305: v41.07,18.36 40.84,18.36 37.88,21.31 36.25,21.31 33.14,24.43 33.14,33.45 v32.98,33.6
SRAM_CS  (via drill 0.51)
  Top 0.254: IC2.1 50.96,26.83 50.41,27.38 44.18,27.38 43.58,26.77 IC3.1 43.56,25.44 43.56,23.65 42.94,23.02 38.58,23.02 36.41,20.85 36.41,19.06 v36.02,18.67 | IC1.55 26.27,31.79 v26.29,31.82
  Bottom 0.254: v36.02,18.67 35.78,18.67 31.89,22.56 31.89,28.16 30.34,29.71 28.86,29.71 26.76,31.82 v26.29,31.82
SWCLK  (via drill 0.51)
  Top 0.254: IC1.49 26.17,34.79 v27.05,33.91
  Bottom 0.254: J1.4 33.05,38.2 28.5,33.5 27.46,33.5 v27.05,33.91
SWDIO  (via drill 0.51)
  Top 0.254: IC1.46 27.46,35.56 27.7,35.32 28.57,35.32 v28.81,35.09
  Bottom 0.254: J1.3 30.5,36.79 v28.81,35.09
SWV33  (via drill 0.51)
  Top 0.305: IC4.4 58.12,26.39 62.59,30.85 J4.3 | IC5.3 42.44,4 v42.47,3.97
  Top 0.61: v28.32,6.84 28.63,6.84
  Bottom 0.61: J4.3 69.96,30.85 71.25,29.56 71.25,7.31 67.91,3.97 v42.47,3.97 31.19,3.97 v28.32,6.84
  pour Top (no thermals): 30.48,7.54 30.48,4.76 27.7,4.76 27.7,7.54
SWV50  (via drill 0.51)
  Top 0.305: IC4.3 58.77,26.26 62.07,29.56 67.52,29.56 67.99,30.03 67.99,32.19 J4.2
  Top 0.61: C16.1 29.63,8.87 30,8.49 37.96,8.49 | 37.96,8.49 38.96,8.49 39.64,7.81 IC5.1 | v37.96,2.18 37.96,8.49
  Bottom 0.61: J4.2 71.78,33.39 73.12,32.05 73.12,6.92 68.38,2.18 v37.96,2.18
  pour Top (no thermals): 30.48,13.34 30.48,9.6 27.7,9.6 27.7,13.34
UART_RX  (via drill 0.51)
  Top 0.254: IC1.43 28.96,37.98 29.33,38.35 29.33,41.69 30.57,42.94 35.47,42.94 v36.09,42.32
  Bottom 0.254: J2.2 57.82,39.88 55.38,42.32 v36.09,42.32
UART_TX  (via drill 0.51)
  Top 0.254: IC1.42 29.46,37.78 31.74,40.06 31.74,41.69 32.52,42.47 34.07,42.47 v35.39,41.15
  Bottom 0.254: v35.39,41.15 53.96,41.15 J2.3
USB_D+  (1 unrouted)
  Top 0.254: IC1.45 27.96,38.25 27.78,38.43 21.16,38.43 14.45,31.72 14.45,26.33 11.47,23.35 R6.1
USB_D-  (1 unrouted)
  Top 0.254: IC1.44 28.46,38.7 28.18,38.99 20.94,38.99 13.97,32.02 13.97,26.57 12.07,24.67 R5.1
USB_DET  (via drill 0.51)
  Top 0.254: IC1.50 23.71,34.29 v23.02,33.6 | R2.2 v13.69,19.91
  Bottom 0.254: v23.02,33.6 23.02,32.75 20.15,29.87 18.59,29.87 16.8,28.08 16.8,26.76 13.69,23.65 v13.69,19.91
USBLED
  Top 0.254: IC1.40 30.46,38.16 31.5,39.2 34.85,39.2 37.1,41.46 R20.2
V33PU  (via drill 0.51)
  Top 0.254: IC6.6 37.65,14.59 | 37.65,14.59 35.1,14.59 v34.87,14.82 | v37.65,11.12 37.65,14.59 | IC1.57 23.09,30.79 v23.02,30.73
  Top 0.305: RN3.7 47.52,10.36 46.83,11.05 43.09,11.05 v43.02,11.12
  Bottom 0.254: v34.87,14.82 34.15,15.54 34.15,16.8 29.91,21.04 29.91,25.8 29.26,26.45 29.26,27.83 26.6,30.49 23.26,30.49 v23.02,30.73
  Bottom 0.305: v43.02,11.12 v37.65,11.12
V50PU  (via drill 0.51)
  Top 0.254: IC5.6 39.98,9.61 | v36.64,13.15 36.64,11.12 38.15,9.61 39.98,9.61 | v39.98,8.87 39.98,9.61 | 23.34,31.43 v23.02,31.74 23.47,31.29 IC1.56
  Top 0.305: RN3.8 44.85,9.69 v44.03,8.87
  Bottom 0.254: v36.64,13.15 36.64,15.01 30.49,21.16 30.49,25.93 29.79,26.63 29.79,28 26.68,31.11 23.65,31.11 v23.02,31.74
  Bottom 0.305: v44.03,8.87 v39.98,8.87
VCC  (16 unrouted)
VCCEXT  (4 unrouted)
VCCIO_2  (1 unrouted)
VCCIO_3  (1 unrouted)
VEXTERN  (via drill 0.51)
  Top 0.305: IC6.3 42.48,12.76 v45.27,12.76 46.58,12.76 RN1.1
  Bottom 0.457: v45.27,12.76 45.27,6.38 45.51,6.14 68.69,6.14 70.16,7.62 70.16,27.23 69.08,28.31 J4.4
VEXTPU  (via drill 0.51)
  Top 0.254: IC7.6 47.59,37.04 47.06,37.57 R21.1 43.87,38.51 36.25,38.51 35.47,37.73 32.13,37.73 31.96,37.56 IC1.37
  Top 0.305: IC7.6 IC7.5 48.24,34.21 v48.38,34.07 48.23,34.23 | IC7.13 IC7.12 49.55,31.19 v49.78,31.43
  Bottom 0.305: v49.78,31.43 49.78,32.67 v48.38,34.07
VPUN  (via drill 0.51)
  Top 0.305: IC7.3 IC7.2 50.2,35.1 v49.78,34.69 | IC7.9 47.59,29.26 47.76,29.09 48.7,29.09 48.9,29.29 IC7.11 48.9,31.94 49.32,32.36 51.03,32.36 v52.04,31.35 | RN1.3 48.32,11.89 v49.01,11.2
  Top 0.406: IC6.4 43.28,14.59 v43.56,14.31
  Bottom 0.305: v49.78,34.69 49.78,33.6 v52.04,31.35
  Bottom 0.406: v52.04,31.35 52.27,31.11 58.5,31.11 58.81,31.43 61.76,31.43 66.12,27.07 68.92,27.07 69.39,26.6 69.39,11.67 68.92,11.2 v49.01,11.2 45.9,14.31 v43.56,14.31
VREGEN  (via drill 0.51)
  Top 0.254: VR2.3 25.4,3.42 25.4,3.41 v25.4,2.54 | 25.4,8.57 VR3.3 25.4,8.54 v25.4,7.62 | R19.2 58.55,46 58.5,46.05 51.65,46.05 49.16,43.56 v44.18,43.56 | 22.58,28.29 IC1.62 21.88,28.29 v21.59,28.57 19.91,30.25 v19.91,31.43 19.21,31.43 18.67,30.88 R1.1 | v25.51,43.72 29.64,43.72 v29.87,43.56
  Bottom 0.254: v25.4,2.54 v25.4,7.62 24.12,7.62 18.05,13.69 18.05,27.38 19.29,28.63 21.54,28.63 v21.59,28.57 | v44.18,43.56 v29.87,43.56 | v19.91,31.43 19.91,42.63 21,43.72 v25.51,43.72
VUSB  (via drill 0.51)  (8 unrouted)
  Top 0.305: IC7.14 50.84,29.01 52.01,27.84 C18.1 52.78,30.07 53.52,30.8 v53.52,32.05 | R13.1 v24.13,15.24 | IC6.5 41.69,14.16 41.23,13.69 40.6,13.69 40.29,13.38 40.29,10.97 | v43.56,3.08 43.56,8.09 42.94,8.71 42.16,8.71 41.69,9.18 IC5.5 41.69,10.19 40.91,10.97 40.29,10.97 | C19.1 40.29,10.97
  Bottom 0.254: 30.52,3.08 30.49,3.11
  Bottom 0.305: v24.13,15.24 24.13,10.72 26.76,8.09 26.76,6.84 30.49,3.11 | v53.52,32.05 53.83,31.74 56.16,31.74 56.63,32.2 70.94,32.2 72.19,30.96 72.19,7.08 68.19,3.08 v43.56,3.08 30.52,3.08
  pour Top (no thermals): 9.68,10.16 17.78,10.16 17.78,15.95 25.4,15.95 25.4,5.08 23.5,5.08 23.5,7.62 9.68,7.62

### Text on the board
tPlace: FEB 2018 | UART | TX | RX | GND | Ian Lesnet | I+S 2018 | v.trocio
bPlace: FEB 2018
tNames: B0 | B1 | PWR | USB | MODE | VREG | 3.3V | GND | SW- / DIO | SW- / CLK | Bus Pirate NG v1.0 | BOOT
bNames: PWR | USB | MODE | VREG | GND | +5V | 3V3 | VPU | ADC/DAC | Bus Pirate NG v1.0 | AUX | CS | MISO | CLK | MOSI | Fulfillment by | Seeed Studio | www.seeedstudio.com
tValues: vimark
Reference: GND | +5v | +3v3 | Vpu | USB | ADC/DAC | I/O header | AUX0 | CS | MISO | CLK | MOSI | BUS PIRATE NG v1.0 | CC-0 | Ian Lesnet FEB 2018 | http://dangerousprototypes.com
